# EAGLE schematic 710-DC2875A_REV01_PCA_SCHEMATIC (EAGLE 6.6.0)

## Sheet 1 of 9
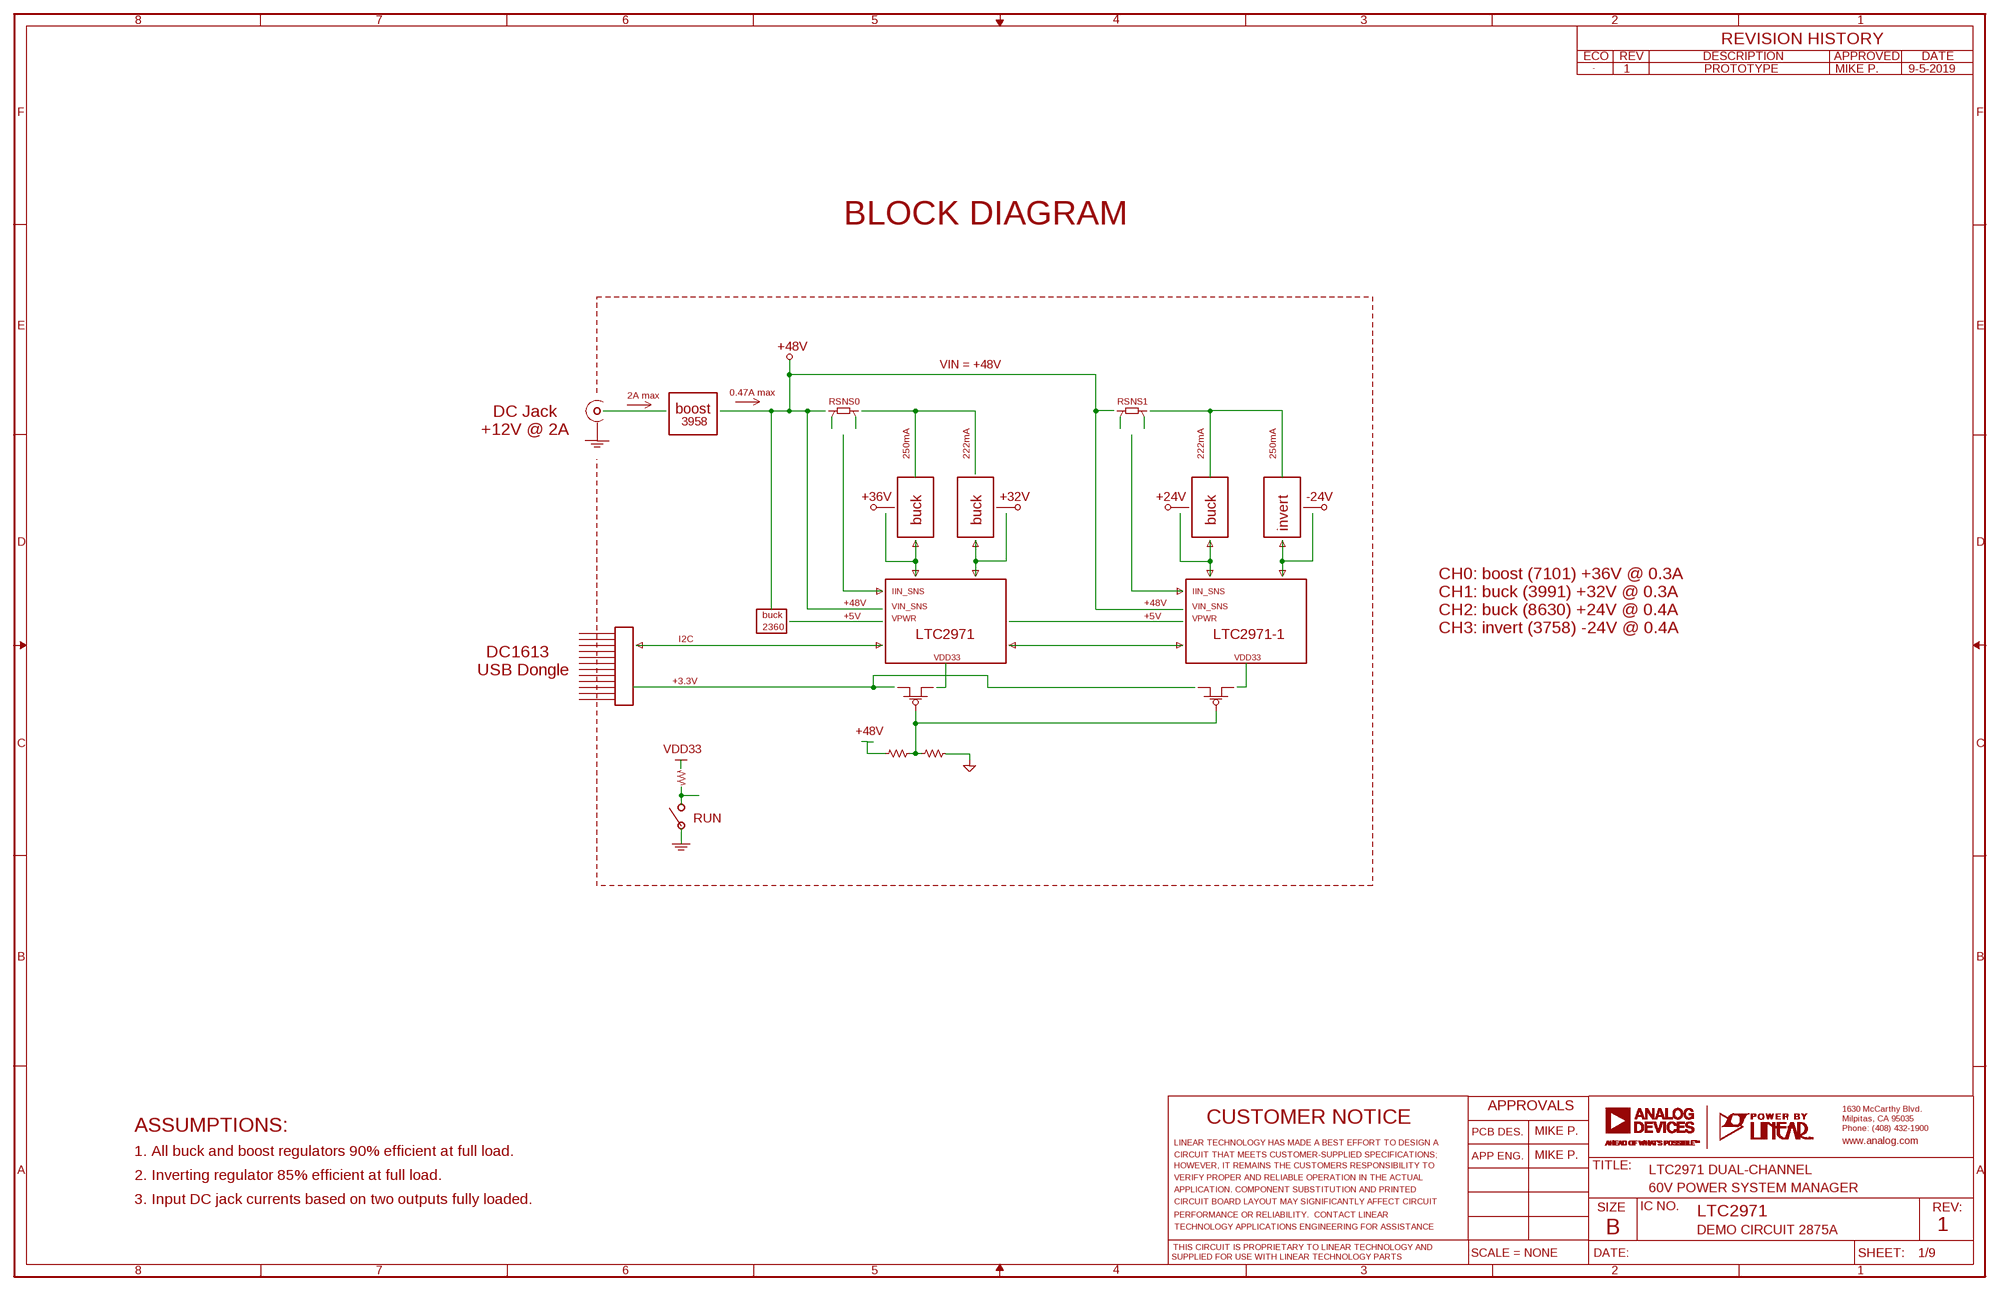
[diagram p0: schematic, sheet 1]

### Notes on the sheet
- 1 | PROTOTYPE | MIKE P. | 9-5-2019
- BLOCK DIAGRAM
- +48V
- VIN = +48V
- 0.47A max
- 2A max
- RSNS0 | RSNS1
- boost
- 3958
- DC Jack
  +12V @ 2A
- 250mA | 222mA | 222mA | 250mA
- +36V | +32V | +24V | -24V
- buck | buck | buck
- invert
- IIN_SNS | IIN_SNS
- +48V | +48V
- VIN_SNS | VIN_SNS
- buck | +5V | +5V
- VPWR | VPWR
- 2360
- CH0: boost (7101) +36V @ 0.3A
  CH1: buck (3991) +32V @ 0.3A
  CH2: buck (8630) +24V @ 0.4A
  CH3: invert (3758) -24V @ 0.4A
- LTC2971 | LTC2971-1
- I2C
- VDD33 | VDD33
- DC1613
  USB Dongle
- +3.3V
- +48V
- VDD33
- RUN
- ASSUMPTIONS: | MIKE P.
- 1. All buck and boost regulators 90% efficient at full load. | MIKE P.
- LTC2971 DUAL-CHANNEL
- 2. Inverting regulator 85% efficient at full load.
- 60V POWER SYSTEM MANAGER
- 3. Input DC jack currents based on two outputs fully loaded.
- LTC2971
- DEMO CIRCUIT 2875A | 1

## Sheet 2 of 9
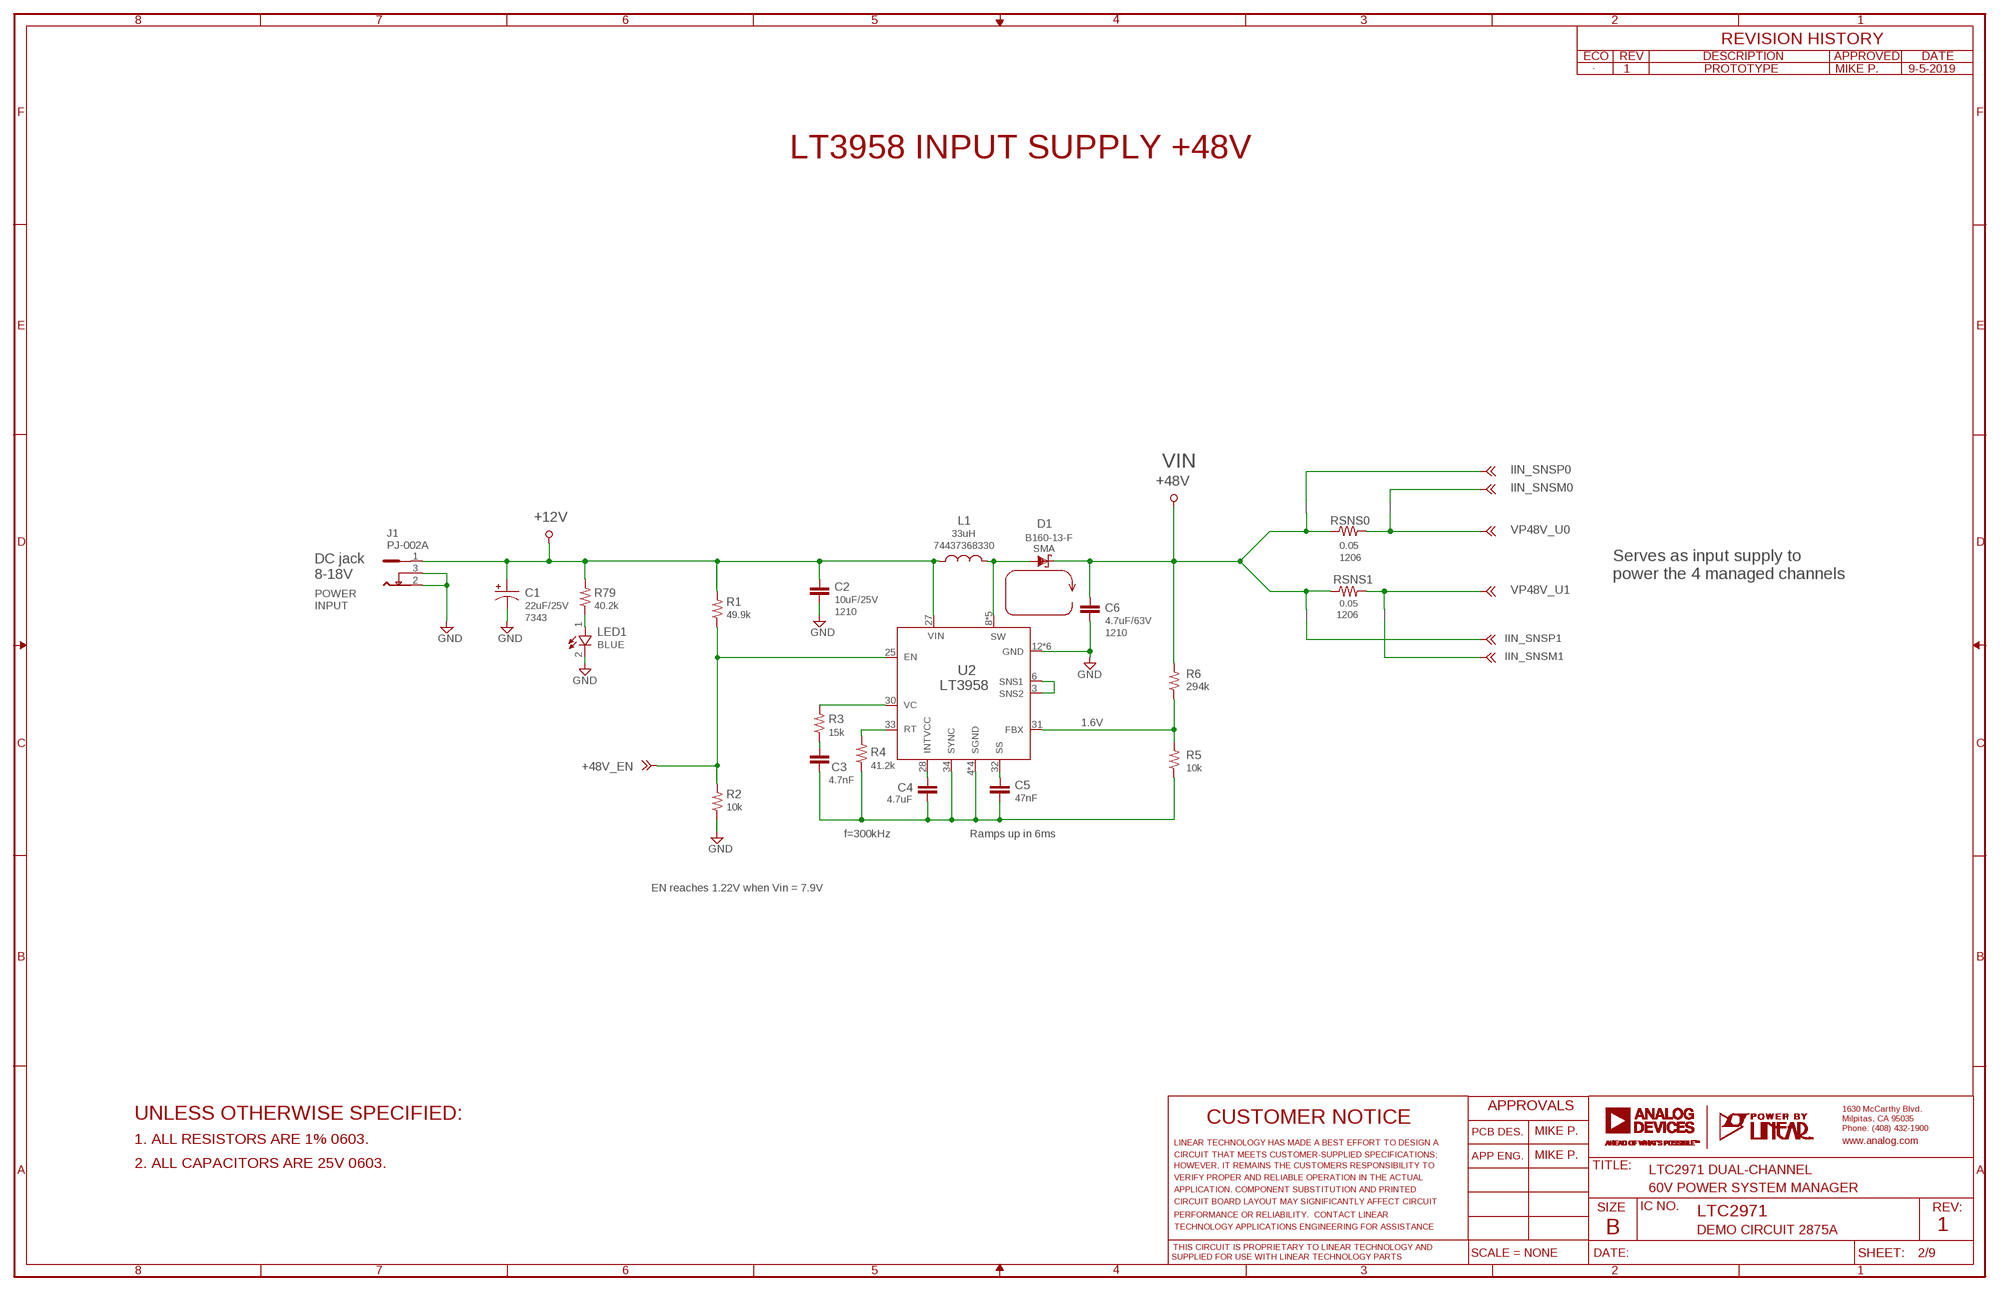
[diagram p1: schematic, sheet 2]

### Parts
C1  22uF/25V  CPOL-US7343  [C7343]
C2  10uF/25V  CC1210_BOX  [C1210_BOX]
C3  4.7nF  CC0603_BOX  [C0603_BOX]
C4  4.7uF  CC0603_BOX  [C0603_BOX]
C5  47nF  CC0603_BOX  [C0603_BOX]
C6  4.7uF/63V  CC1210_BOX  [C1210_BOX]
D1  B160-13-F  SCHOTTKY-DIODESMA  [SMA]
J1  PJ-002A  [PJ-002A/B]
L1  33uH  LWE-LHMI-10  [WE-LHMI-10]
LED1  BLUE  LED-0603  [CHIPLED_0603]
NB12  NODE_BREAKER_BOT  [NODE_BREAKER_BOT]
NB13  NODE_BREAKER_BOT  [NODE_BREAKER_BOT]
NB17  NODE_BREAKER_BOT  [NODE_BREAKER_BOT]
NB18  NODE_BREAKER_BOT  [NODE_BREAKER_BOT]
R1  49.9k  RR0603_BOX  [R0603_BOX]
R2  10k  RR0603_BOX  [R0603_BOX]
R3  15k  RR0603_BOX  [R0603_BOX]
R4  41.2k  RR0603_BOX  [R0603_BOX]
R5  10k  RR0603_BOX  [R0603_BOX]
R6  294k  RR0603_BOX  [R0603_BOX]
R79  40.2k  RR0603_BOX  [R0603_BOX]
RSNS0  0.05  RR1206_BOX  [R1206_BOX]
RSNS1  0.05  RR1206_BOX  [R1206_BOX]
TP14  +12V  TURRET_LARGE_2501  [TURRET_LARGE_2501]
TP15  +48V  TURRET_LARGE_2501  [TURRET_LARGE_2501]
TP36  TESPOINT_SMD  TESTPOINT_SMDVIA  [VIA]
U2  LT3958  [QFN36-5X6]

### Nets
+12V: C1.+ C2.1 J1.1 L1.1 R1.2 R79.2 TP14.TP U2.27(VIN) ; also sheet 9
+48V [HV]: C6.1 D1.C NB12.1 NB17.1 R6.2 RSNS0.1 RSNS1.1 TP15.TP ; also sheet 5
+48V_EN: R1.1 R2.2 TP36.1 U2.25(EN)
GND: C1.- C2.2 C6.2 J1.2 J1.3 LED1.C R2.1 U2.12(GND) U2.13(GND) U2.14(GND) U2.15(GND) U2.16(GND) U2.17(GND) ; also sheet 3,4,5,6,7,8,9
IIN_SNSM0 [HV]: NB13.2 ; also sheet 5
IIN_SNSM1 [HV]: NB18.2 ; also sheet 8
IIN_SNSP0 [HV]: NB12.2 ; also sheet 5
IIN_SNSP1 [HV]: NB17.2 ; also sheet 8
N$8: C4.1 U2.28(INTVCC)
N$12: LED1.A R79.1
N$13: U2.3(SNS2) U2.6(SNS1)
N$18: R3.2 U2.30(VC)
N$21: C5.1 U2.32(SS)
N$30 [HV]: D1.A L1.2 U2.8(SW) U2.9(SW) U2.20(SW) U2.21(SW) U2.38(SW)
N$32: R4.2 U2.33(RT)
N$51: R5.2 R6.1 U2.31(FBX)
N$61: C3.1 R3.1
SGND: C3.2 C4.2 C5.2 R4.1 R5.1 U2.4(SGND) U2.23(SGND) U2.24(SGND) U2.34(SYNC) U2.37(SGND)
VP48V_U0 [HV]: NB13.1 RSNS0.2 ; also sheet 3,4,5
VP48V_U1 [HV]: NB18.1 RSNS1.2 ; also sheet 6,7,8

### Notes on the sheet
- 1 | PROTOTYPE | MIKE P. | 9-5-2019
- LT3958 INPUT SUPPLY +48V
- VIN
- 74437368330
- SMA
- 1206
- DC jack
  8-18V
- Serves as input supply to 
  power the 4 managed channels
- POWER
  INPUT
- 1210
- 1206
- 7343
- 1210
- 1.6V
- f=300kHz | Ramps up in 6ms
- EN reaches 1.22V when Vin = 7.9V
- UNLESS OTHERWISE SPECIFIED:
- MIKE P.
- 1. ALL RESISTORS ARE 1% 0603.
- MIKE P.
- 2. ALL CAPACITORS ARE 25V 0603.
- LTC2971 DUAL-CHANNEL
- 60V POWER SYSTEM MANAGER
- LTC2971
- DEMO CIRCUIT 2875A | 1

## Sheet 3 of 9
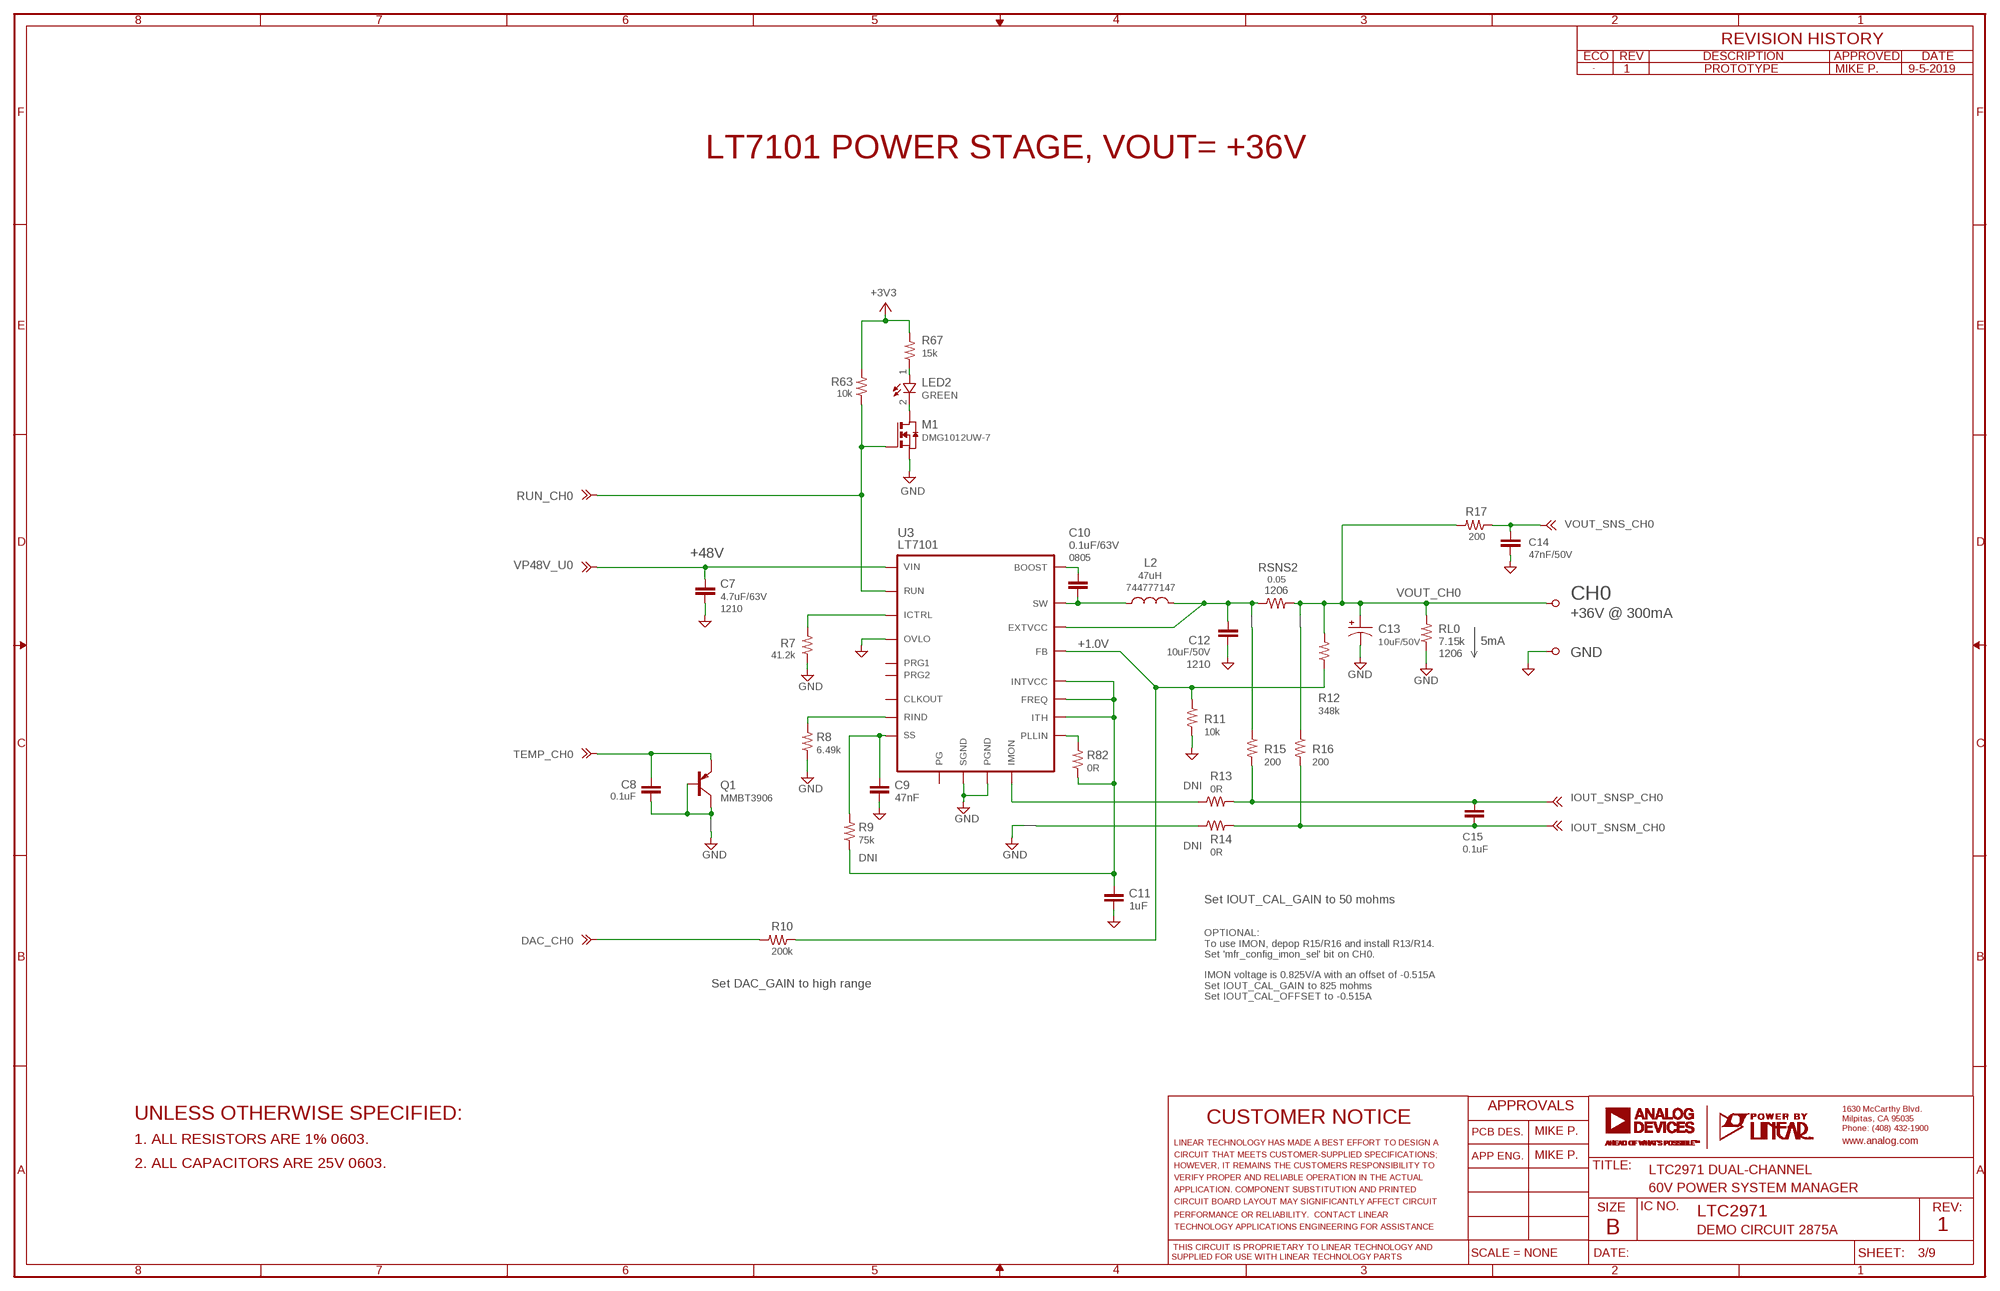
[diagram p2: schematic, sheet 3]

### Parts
C7  4.7uF/63V  CC1210_BOX  [C1210_BOX]
C8  0.1uF  CC0603_BOX  [C0603_BOX]
C9  47nF  CC0603_BOX  [C0603_BOX]
C10  0.1uF/63V  CC0805_BOX  [C0805_BOX]
C11  1uF  CC0603_BOX  [C0603_BOX]
C12  10uF/50V  CC1210_BOX  [C1210_BOX]
C13  10uF/50V  CPOL-USUD-6,3X5,8  [UD-6,3X5,8_NICHICON]
C14  47nF/50V  CC0603_BOX  [C0603_BOX]
C15  0.1uF  CC0603_BOX  [C0603_BOX]
L2  47uH  LWE-PD-7.3  [WE-PD-7.3]
LED2  GREEN  LED-0603  [CHIPLED_0603]
M1  DMG1012UW-7  NCH(SOT323)  [SOT323]
NB5  NODE_BREAKER  [NODE_BREAKER]
NB19  NODE_BREAKER  [NODE_BREAKER]
NB20  NODE_BREAKER  [NODE_BREAKER]
NB21  NODE_BREAKER  [NODE_BREAKER]
Q1  MMBT3906  PNP  [SC70]
R7  41.2k  RR0603_BOX  [R0603_BOX]
R8  6.49k  RR0603_BOX  [R0603_BOX]
R9  75k  RR0603_BOX  [R0603_BOX]
R10  200k  RR0603_BOX  [R0603_BOX]
R11  10k  RR0603_BOX  [R0603_BOX]
R12  348k  RR0603_BOX  [R0603_BOX]
R13  0R  RR0603_BOX  [R0603_BOX]
R14  0R  RR0603_BOX  [R0603_BOX]
R15  200  RR0603_BOX  [R0603_BOX]
R16  200  RR0603_BOX  [R0603_BOX]
R17  200  RR0603_BOX  [R0603_BOX]
R63  10k  RR0603_BOX  [R0603_BOX]
R67  15k  RR0603_BOX  [R0603_BOX]
R82  0R  RR0603_BOX  [R0603_BOX]
RL0  7.15k  RR1206_BOX  [R1206_BOX]
RSNS2  0.05  RR1206_BOX  [R1206_BOX]
TP0  CH0  TURRET_LARGE_2501  [TURRET_LARGE_2501]
TP20  TURRET_SMALL_2308  [TURRET_SMALL_2308]
TP24  TESPOINT_SMD  TESTPOINT_SMDVIA  [VIA]
TP25  TESPOINT_SMD  TESTPOINT_SMDVIA  [VIA]
TP26  TESPOINT_SMD  TESTPOINT_SMDVIA  [VIA]
U3  LT7101  [QFN36-5X6-UHE]

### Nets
DAC_CH0: R10.2 TP26.1 ; also sheet 5
GND: C7.2 C9.2 C11.2 C12.2 C13.- C14.2 M1.2(S) NB5.1 NB19.2 R7.1 R8.1 R11.2 RL0.1 TP20.TP1 U3.6(SGND) U3.7(OVLO) U3.35(PGND) U3.36(PGND) U3.37(PGND) ; also sheet 2,4,5,6,7,8,9
INTVCC: C11.1 R9.1 R82.1 U3.9(ITH) U3.11(FREQ) U3.21(INTVCC)
IOUT_SNSM_CH0 [HV]: C15.2 R14.2 R16.2 ; also sheet 5
IOUT_SNSP_CH0 [HV]: C15.1 R13.2 R15.2 ; also sheet 5
N$4: R7.2 U3.16(ICTRL)
N$6: LED2.C M1.3(D)
N$7: LED2.A R67.1
N$20: R8.2 U3.8(RIND)
N$64: C8.2 NB5.2 Q1.1(B) Q1.3(C)
N$73: C9.1 R9.2 U3.15(SS)
N$75 [HV]: R13.1 U3.17(IMON)
N$78 [HV]: C12.1 L2.2 NB20.2 RSNS2.1 U3.20(EXTVCC)
N$94: NB20.1 R15.1
N$98 [HV]: NB19.1 R14.1
N$99: NB21.1 R16.1
N$100: C10.2 L2.1 U3.24(SW) U3.25(SW) U3.26(SW)
N$114: C10.1 U3.27(BOOST)
N$116: R82.2 U3.12(PLLIN)
RUN_CH0: M1.1(G) R63.1 TP24.1 U3.3(RUN) ; also sheet 5
TEMP_CH0: C8.1 Q1.2(E) TP25.1 ; also sheet 5
VDD33_A: R63.2 R67.2 ; supply symbol labelled +3V3 ; also sheet 4,5,6,9
VFB0: R10.1 R11.1 R12.1 U3.10(FB)
VOUT_CH0 [HV]: C13.+ NB21.2 R12.2 R17.2 RL0.2 RSNS2.2 TP0.TP
VOUT_SNS_CH0 [HV]: C14.1 R17.1 ; also sheet 5
VP48V_U0 [HV]: C7.1 U3.30(VIN) U3.31(VIN) U3.32(VIN) ; also sheet 2,4,5
Unconnected: U3.13(CLKOUT) U3.14(PGOOD) U3.18(PRG1) U3.19(PRG2)

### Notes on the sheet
- 1 | PROTOTYPE | MIKE P. | 9-5-2019
- LT7101 POWER STAGE, VOUT= +36V
- +48V
- 0805
- 744777147
- 1206
- CH0
- 1210
- +36V @ 300mA
- +1.0V | 5mA
- 1210 | 1206
- DNI
- DNI
- DNI
- Set IOUT_CAL_GAIN to 50 mohms
- OPTIONAL:
  To use IMON, depop R15/R16 and install R13/R14.
  Set 'mfr_config_imon_sel' bit on CH0.
- Set DAC_GAIN to high range
- IMON voltage is 0.825V/A with an offset of -0.515A
  Set IOUT_CAL_GAIN to 825 mohms
  Set IOUT_CAL_OFFSET to -0.515A
- UNLESS OTHERWISE SPECIFIED:
- MIKE P.
- 1. ALL RESISTORS ARE 1% 0603.
- MIKE P.
- 2. ALL CAPACITORS ARE 25V 0603.
- LTC2971 DUAL-CHANNEL
- 60V POWER SYSTEM MANAGER
- LTC2971
- DEMO CIRCUIT 2875A | 1

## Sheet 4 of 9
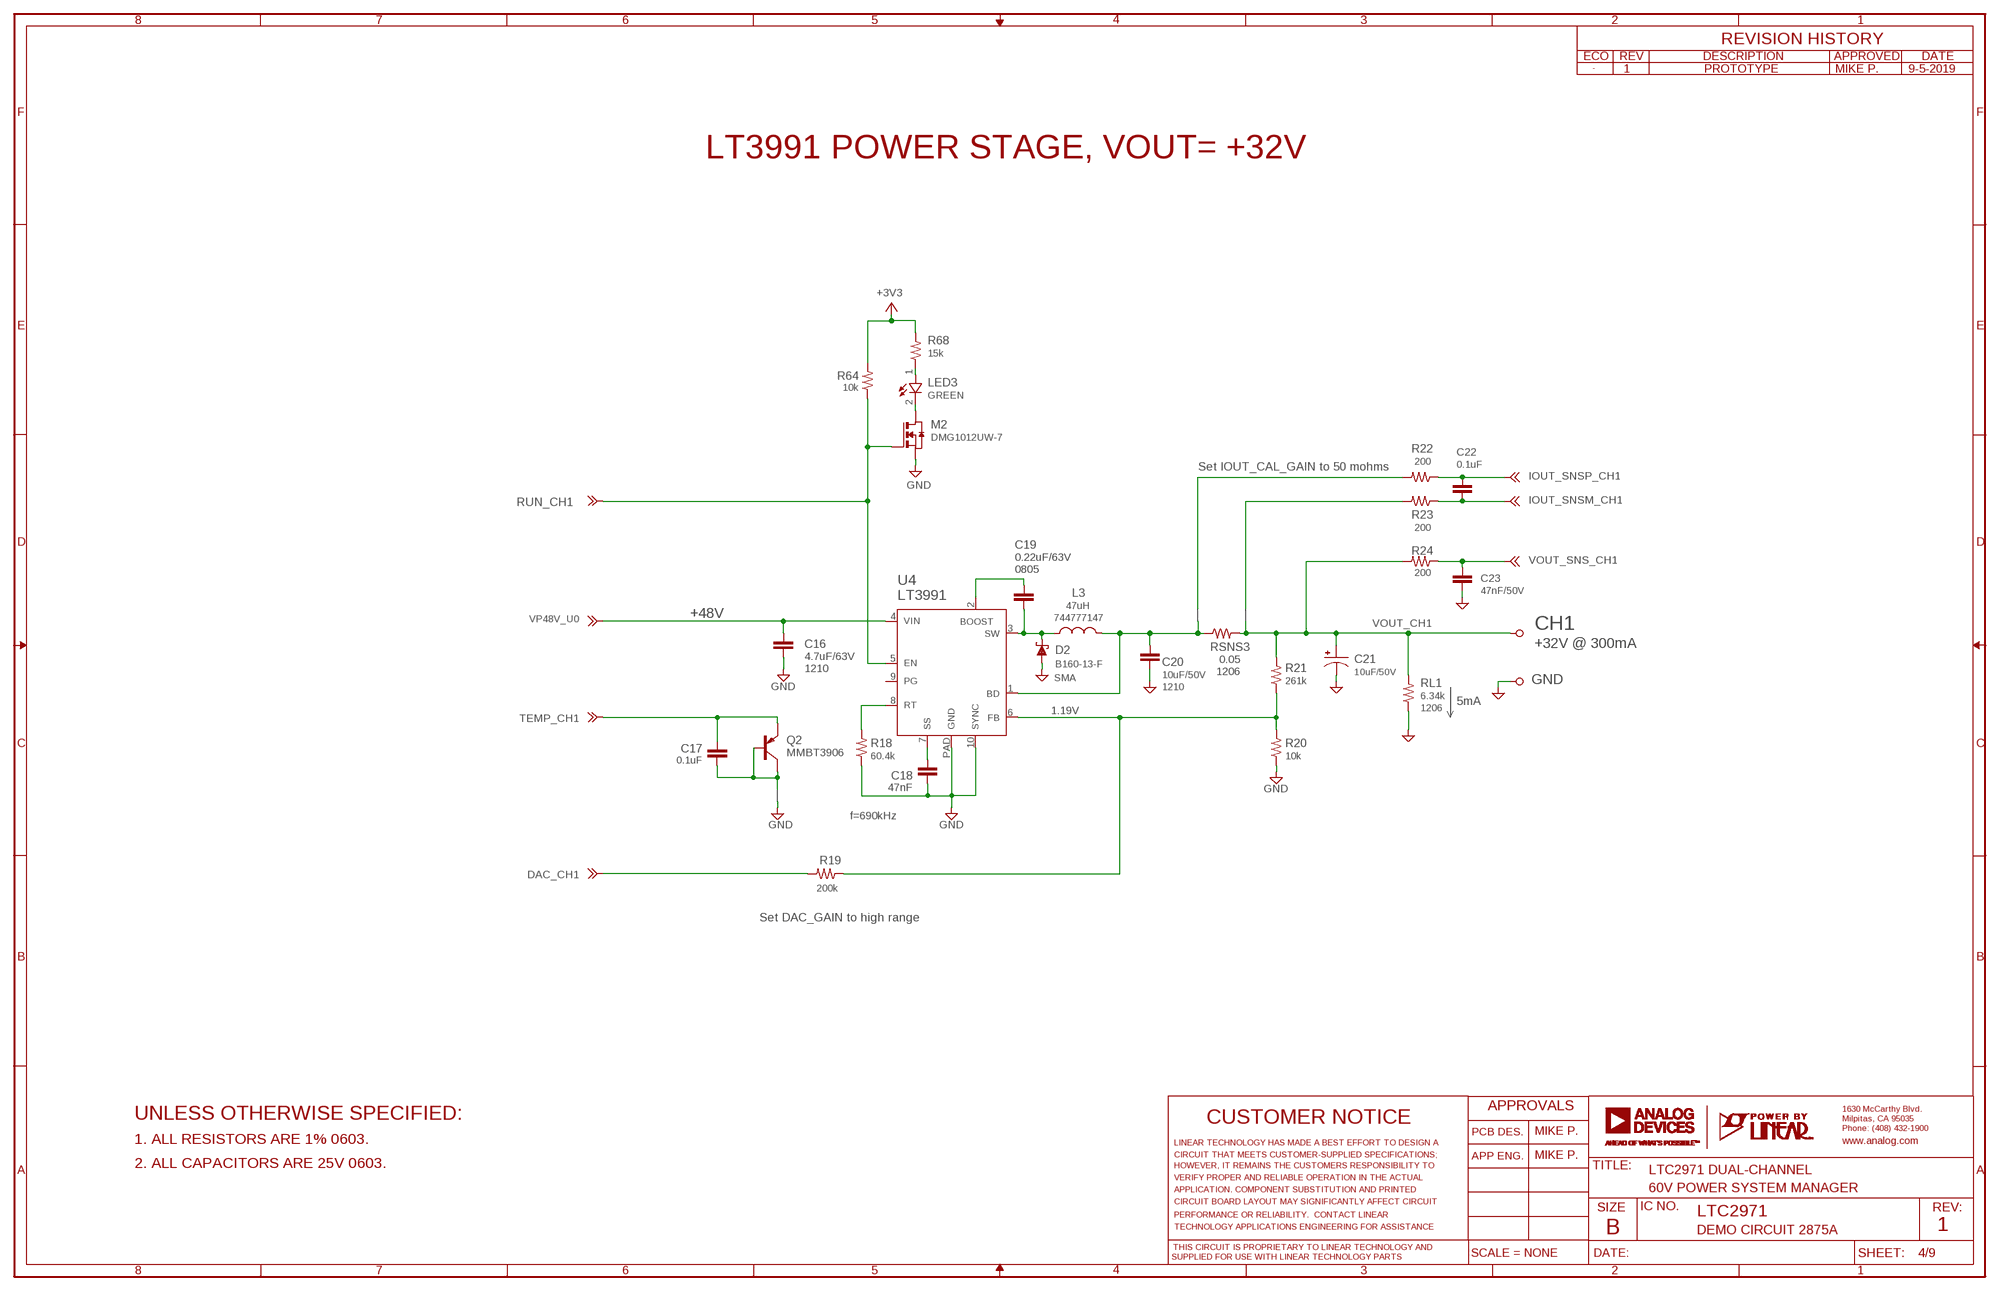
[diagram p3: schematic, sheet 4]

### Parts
C16  4.7uF/63V  CC1210_BOX  [C1210_BOX]
C17  0.1uF  CC0603_BOX  [C0603_BOX]
C18  47nF  CC0603_BOX  [C0603_BOX]
C19  0.22uF/63V  CC0805_BOX  [C0805_BOX]
C20  10uF/50V  CC1210_BOX  [C1210_BOX]
C21  10uF/50V  CPOL-USUD-6,3X5,8  [UD-6,3X5,8_NICHICON]
C22  0.1uF  CC0603_BOX  [C0603_BOX]
C23  47nF/50V  CC0603_BOX  [C0603_BOX]
D2  B160-13-F  SCHOTTKY-DIODESMA  [SMA]
L3  47uH  LWE-PD-7.3  [WE-PD-7.3]
LED3  GREEN  LED-0603  [CHIPLED_0603]
M2  DMG1012UW-7  NCH(SOT323)  [SOT323]
NB3  NODE_BREAKER  [NODE_BREAKER]
NB4  NODE_BREAKER  [NODE_BREAKER]
NB14  NODE_BREAKER  [NODE_BREAKER]
Q2  MMBT3906  PNP  [SC70]
R18  60.4k  RR0603_BOX  [R0603_BOX]
R19  200k  RR0603_BOX  [R0603_BOX]
R20  10k  RR0603_BOX  [R0603_BOX]
R21  261k  RR0603_BOX  [R0603_BOX]
R22  200  RR0603_BOX  [R0603_BOX]
R23  200  RR0603_BOX  [R0603_BOX]
R24  200  RR0603_BOX  [R0603_BOX]
R64  10k  RR0603_BOX  [R0603_BOX]
R68  15k  RR0603_BOX  [R0603_BOX]
RL1  6.34k  RR1206_BOX  [R1206_BOX]
RSNS3  0.05  RR1206_BOX  [R1206_BOX]
TP1  CH1  TURRET_LARGE_2501  [TURRET_LARGE_2501]
TP21  TURRET_SMALL_2308  [TURRET_SMALL_2308]
TP27  TESPOINT_SMD  TESTPOINT_SMDVIA  [VIA]
TP28  TESPOINT_SMD  TESTPOINT_SMDVIA  [VIA]
TP29  TESPOINT_SMD  TESTPOINT_SMDVIA  [VIA]
U4  LT3991  [MSOP10_EXP]

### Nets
DAC_CH1: R19.2 TP29.1 ; also sheet 5
GND: C16.2 C18.2 C20.2 C21.- C23.2 D2.A M2.2(S) NB14.1 R18.1 R20.1 RL1.1 TP21.TP1 U4.10(SYNC) U4.PAD(GND) ; also sheet 2,3,5,6,7,8,9
IOUT_SNSM_CH1 [HV]: C22.2 R23.1 ; also sheet 5
IOUT_SNSP_CH1 [HV]: C22.1 R22.1 ; also sheet 5
N$10: LED3.C M2.3(D)
N$11: LED3.A R68.1
N$33: R18.2 U4.8(RT)
N$36 [HV]: C20.1 L3.2 NB3.1 RSNS3.1 U4.1(BD)
N$59: C18.1 U4.7(SS)
N$67: C17.2 NB14.2 Q2.1(B) Q2.3(C)
N$70: C19.2 D2.C L3.1 U4.3(SW)
N$71: C19.1 U4.2(BOOST)
N$300 [HV]: NB3.2 R22.2
N$301 [HV]: NB4.2 R23.2
RUN_CH1: M2.1(G) R64.1 TP27.1 U4.5(EN) ; also sheet 5
TEMP_CH1: C17.1 Q2.2(E) TP28.1 ; also sheet 5
VDD33_A: R64.2 R68.2 ; supply symbol labelled +3V3 ; also sheet 3,5,6,9
VFB1: R19.1 R20.2 R21.1 U4.6(FB)
VOUT_CH1 [HV]: C21.+ NB4.1 R21.2 R24.2 RL1.2 RSNS3.2 TP1.TP
VOUT_SNS_CH1 [HV]: C23.1 R24.1 ; also sheet 5
VP48V_U0 [HV]: C16.1 U4.4(VIN) ; also sheet 2,3,5
Unconnected: U4.9(PG)

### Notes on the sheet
- 1 | PROTOTYPE | MIKE P. | 9-5-2019
- LT3991 POWER STAGE, VOUT= +32V
- Set IOUT_CAL_GAIN to 50 mohms
- 0805
- +48V
- 744777147
- CH1
- +32V @ 300mA
- 1210 | 1206
- SMA
- 1210
- 5mA
- 1206
- 1.19V
- f=690kHz
- Set DAC_GAIN to high range
- UNLESS OTHERWISE SPECIFIED:
- MIKE P.
- 1. ALL RESISTORS ARE 1% 0603.
- MIKE P.
- 2. ALL CAPACITORS ARE 25V 0603.
- LTC2971 DUAL-CHANNEL
- 60V POWER SYSTEM MANAGER
- LTC2971
- DEMO CIRCUIT 2875A | 1

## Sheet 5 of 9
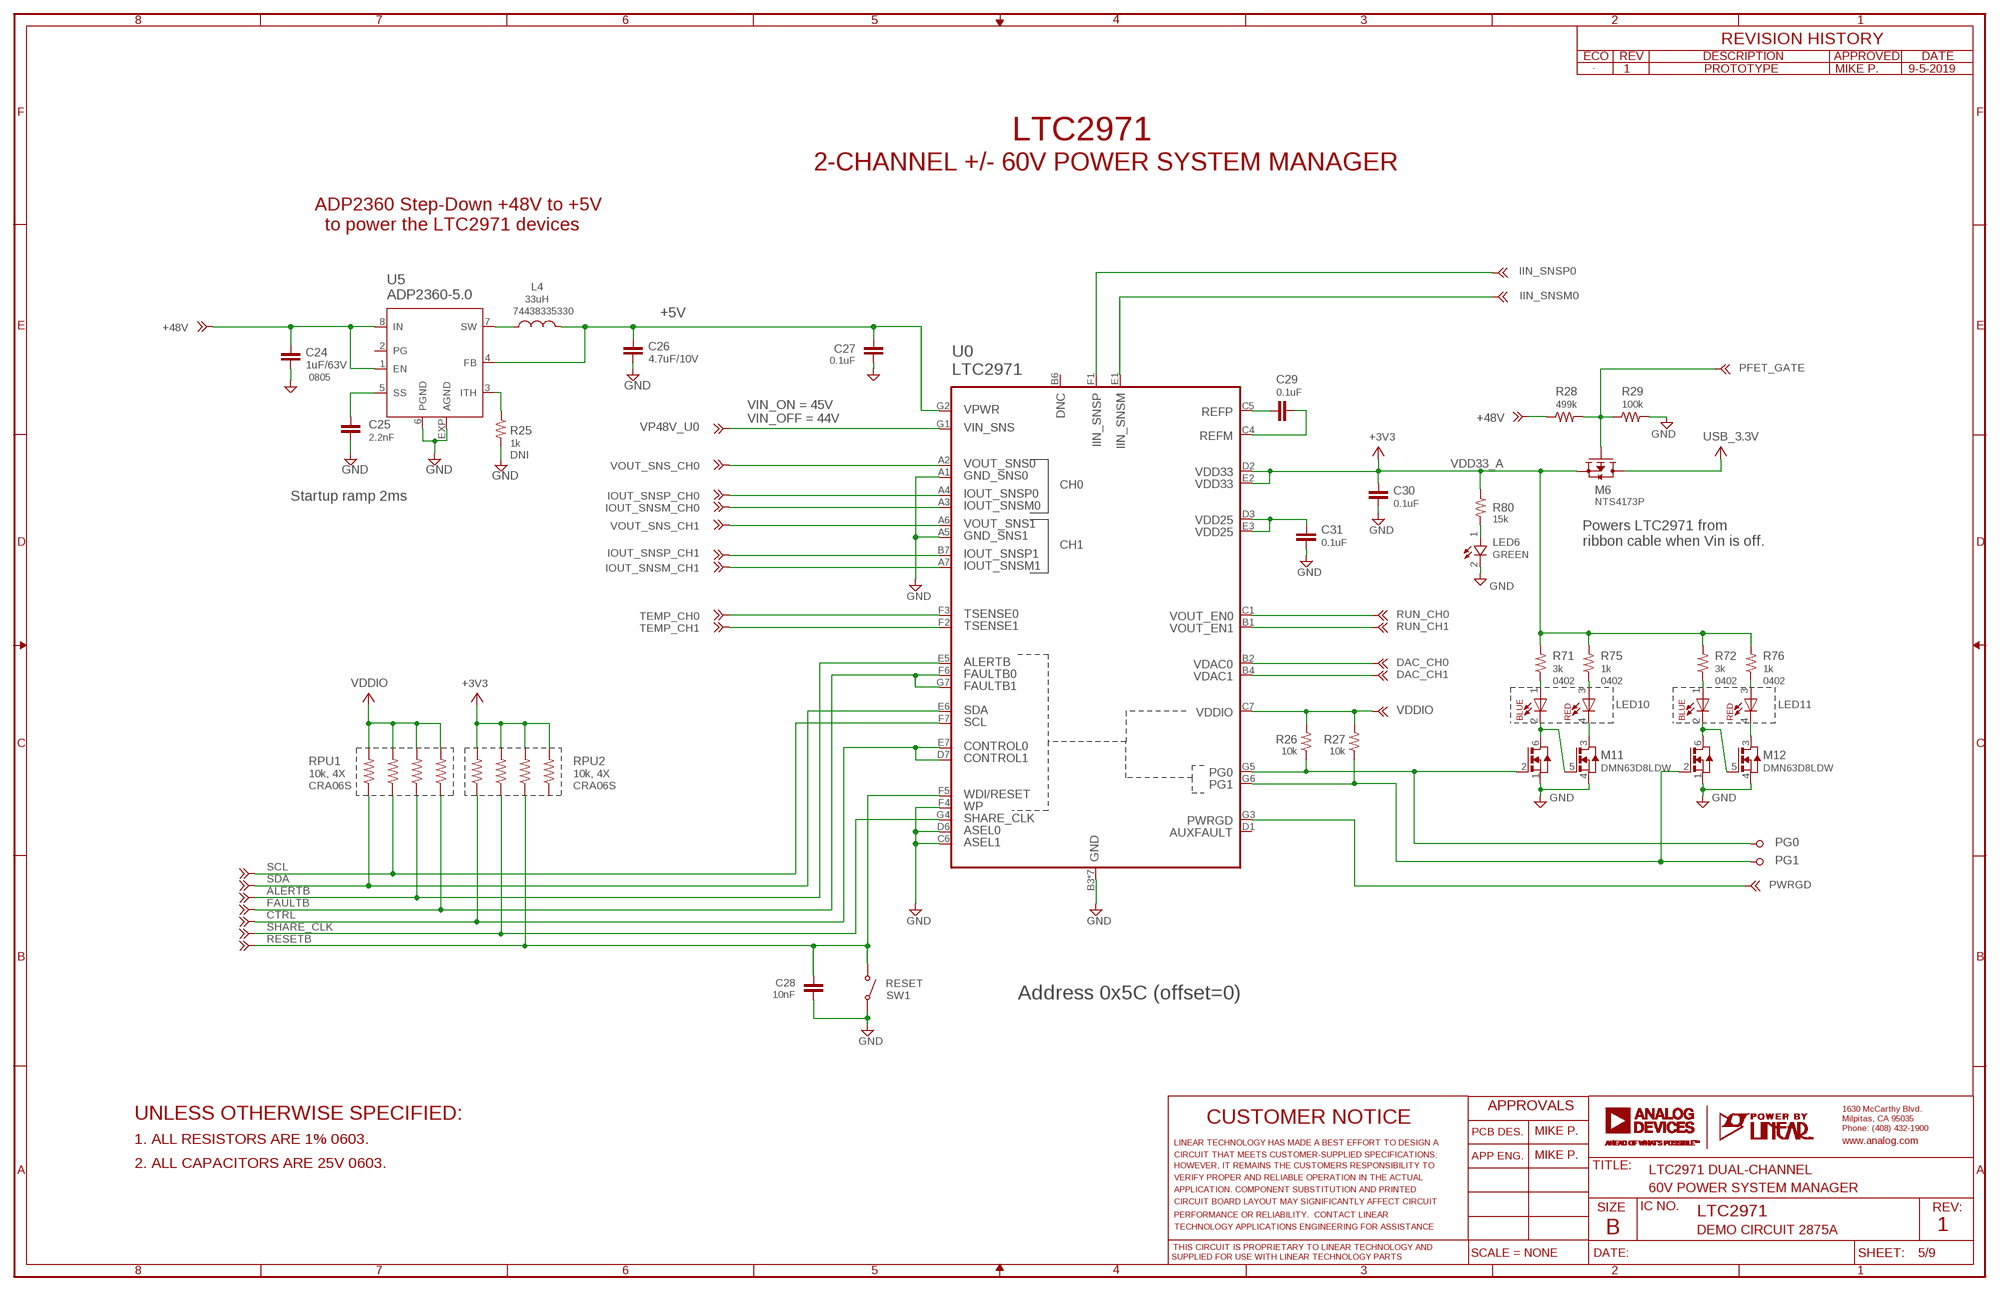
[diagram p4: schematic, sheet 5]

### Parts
C24  1uF/63V  CC0805_BOX  [C0805_BOX]
C25  2.2nF  CC0603_BOX  [C0603_BOX]
C26  4.7uF/10V  CC0603_BOX  [C0603_BOX]
C27  0.1uF  CC0603_BOX  [C0603_BOX]
C28  10nF  CC0603_BOX  [C0603_BOX]
C29  0.1uF  CC0603_BOX  [C0603_BOX]
C30  0.1uF  CC0603_BOX  [C0603_BOX]
C31  0.1uF  CC0603_BOX  [C0603_BOX]
L4  33uH  LWE-MAPI-3.0  [WE-MAPI-3015]
LED6  GREEN  LED-0603  [CHIPLED_0603]
LED10  LED-DUAL-COLOR-BL-RD  [LED-DUAL_1.6X0.8MM]
LED11  LED-DUAL-COLOR-BL-RD  [LED-DUAL_1.6X0.8MM]
M6  NTS4173P  PCH(SOT323)  [SOT323]
M11  DMN63D8LDW  NCH_DUAL_REVERSIBLE  [SOT-363]
M12  DMN63D8LDW  NCH_DUAL_REVERSIBLE  [SOT-363]
R25  1k  RR0603_BOX  [R0603_BOX]
R26  10k  RR0603_BOX  [R0603_BOX]
R27  10k  RR0603_BOX  [R0603_BOX]
R28  499k  RR0603_BOX  [R0603_BOX]
R29  100k  RR0603_BOX  [R0603_BOX]
R71  3k  RR0402_BOX  [R0402_BOX]
R72  3k  RR0402_BOX  [R0402_BOX]
R75  1k  RR0402_BOX  [R0402_BOX]
R76  1k  RR0402_BOX  [R0402_BOX]
R80  15k  RR0603_BOX  [R0603_BOX]
RPU1  10k, 4X  R_ARRAY_4X_CRA06S  [R_VISHAY_CRA06S]
RPU2  10k, 4X  R_ARRAY_4X_CRA06S  [R_VISHAY_CRA06S]
SW1  RS-282G05A3-SM RT  SWITCH_PTS635  [SWITCH_PTS635]
TP16  PG1  TURRET_SMALL_2308  [TURRET_SMALL_2308]
TP17  PG0  TURRET_SMALL_2308  [TURRET_SMALL_2308]
U0  LTC2971  [BGA49]
U5  ADP2360-5.0  ADP2360  [LFCSP8]

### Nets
+48V [HV]: C24.1 R28.1 U5.1(EN) U5.8(VIN) ; also sheet 2
ALERTB: RPU1.R3_1 U0.E5(ALERTB) ; also sheet 8,9
CTRL: RPU2.R1_1 U0.D7(CTRL1) U0.E7(CTRL0) ; also sheet 8,9
DAC_CH0: U0.B2(VDAC0) ; also sheet 3
DAC_CH1: U0.B4(VDAC1) ; also sheet 4
FAULTB: RPU1.R4_1 U0.F6(FAULTB0) U0.G7(FAULTB1) ; also sheet 8,9
GND: C24.2 C25.2 C26.2 C27.1 C28.1 C30.2 C31.1 LED6.C M11.1(S1) M11.4(S2) M12.1(S1) M12.4(S2) R25.2 R29.2 SW1.SW2 U0.A1(GND_SNS0) U0.A5(GND_SNS1) U0.B3(GND) U0.B5(GND) U0.C2(GND) U0.C3(GND) U0.C6(ASEL1) U0.D4(GND) U0.D5(GND) U0.D6(ASEL0) U0.E4(GND) U0.F4(WP) U5.6(PGND) U5.EXP(AGND) ; also sheet 2,3,4,6,7,8,9
IIN_SNSM0 [HV]: U0.E1(IIN_SNSM) ; also sheet 2
IIN_SNSP0 [HV]: U0.F1(IIN_SNSP) ; also sheet 2
IOUT_SNSM_CH0 [HV]: U0.A3(IOUT_SNSM0) ; also sheet 3
IOUT_SNSM_CH1 [HV]: U0.A7(IOUT_SNSM1) ; also sheet 4
IOUT_SNSP_CH0 [HV]: U0.A4(IOUT_SNSP0) ; also sheet 3
IOUT_SNSP_CH1 [HV]: U0.B7(IOUT_SNSP1) ; also sheet 4
N$23: C25.1 U5.5(SS)
N$28: LED11.2(C2) M12.5(G2) M12.6(D1)
N$46: L4.1 U5.7(SW)
N$48: R25.1 U5.3(ITH)
N$49: C29.2 U0.C4(REFM)
N$52: C31.2 U0.D3(VDD25_IO) U0.E3(VDD25_IN)
N$53: C29.1 U0.C5(REFP)
N$56: LED11.1(A1) R72.1
N$57: LED11.4(C4) M12.3(D2)
N$58: LED10.1(A1) R71.1
N$60: LED10.3(A3) R75.1
N$63: LED6.A R80.2
N$82: LED10.2(C2) M11.5(G2) M11.6(D1)
N$83: LED11.3(A3) R76.1
N$96: LED10.4(C4) M11.3(D2)
PFET_GATE: M6.1(G) R28.2 R29.1 ; also sheet 8
PG0: M11.2(G1) R26.1 TP16.TP1 U0.G5(PG0)
PG1: M12.2(G1) R27.1 TP17.TP1 U0.G6(PG1)
PWRGD: U0.G3(PWRGD) ; also sheet 8,9
RESETB: C28.2 RPU2.R3_1 SW1.SW1 U0.F5(WDI-RESET) ; also sheet 8,9
RUN_CH0: U0.C1(VOUT_EN0) ; also sheet 3
RUN_CH1: U0.B1(VOUT_EN1) ; also sheet 4
SCL: RPU1.R2_1 U0.F7(SCL) ; also sheet 8,9
SDA: RPU1.R1_1 U0.E6(SDA) ; also sheet 8,9
SHARE_CLK: RPU2.R2_1 U0.G4(SHARE_CLK) ; also sheet 8,9
TEMP_CH0: U0.F3(TSENSE0) ; also sheet 3
TEMP_CH1: U0.F2(TSENSE1) ; also sheet 4
USB_3.3V: M6.3(D) ; supply symbol labelled +3V3 ; also sheet 8,9
VDD33_A: C30.1 M6.2(S) R71.2 R72.2 R75.2 R76.2 R80.1 RPU2.R1_2 RPU2.R2_2 RPU2.R3_2 RPU2.R4_2 U0.D2(VDD33_IO) U0.E2(VDD33_IN) ; supply symbol labelled +3V3 ; also sheet 3,4,6,9
VDDIO: R26.2 R27.2 RPU1.R1_2 RPU1.R2_2 RPU1.R3_2 RPU1.R4_2 U0.C7(VDDIO) ; supply symbol labelled +3V3 ; also sheet 8,9
VOUT_SNS_CH0 [HV]: U0.A2(VOUT_SNS0) ; also sheet 3
VOUT_SNS_CH1 [HV]: U0.A6(VOUT_SNS1) ; also sheet 4
VP5P0: C26.1 C27.2 L4.2 U0.G2(VPWR) U5.4(FB) ; also sheet 8
VP48V_U0 [HV]: U0.G1(VIN_SNS) ; also sheet 2,3,4
Unconnected: RPU2.R4_1 U0.B6(DNC) U0.D1(AUXFAULT) U5.2(PG)

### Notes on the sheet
- 1 | PROTOTYPE | MIKE P. | 9-5-2019
- LTC2971
- 2-CHANNEL +/- 60V POWER SYSTEM MANAGER
- ADP2360 Step-Down +48V to +5V
    to power the LTC2971 devices
- 74438335330
- +5V
- 0805
- VIN_ON = 45V
  VIN_OFF = 44V
- DNI
- Startup ramp 2ms
- Powers LTC2971 from 
  ribbon cable when Vin is off.
- 0402 | 0402 | 0402 | 0402
- CRA06S | CRA06S
- RESET
- Address 0x5C (offset=0)
- UNLESS OTHERWISE SPECIFIED:
- MIKE P.
- 1. ALL RESISTORS ARE 1% 0603.
- MIKE P.
- 2. ALL CAPACITORS ARE 25V 0603.
- LTC2971 DUAL-CHANNEL
- 60V POWER SYSTEM MANAGER
- LTC2971
- DEMO CIRCUIT 2875A | 1

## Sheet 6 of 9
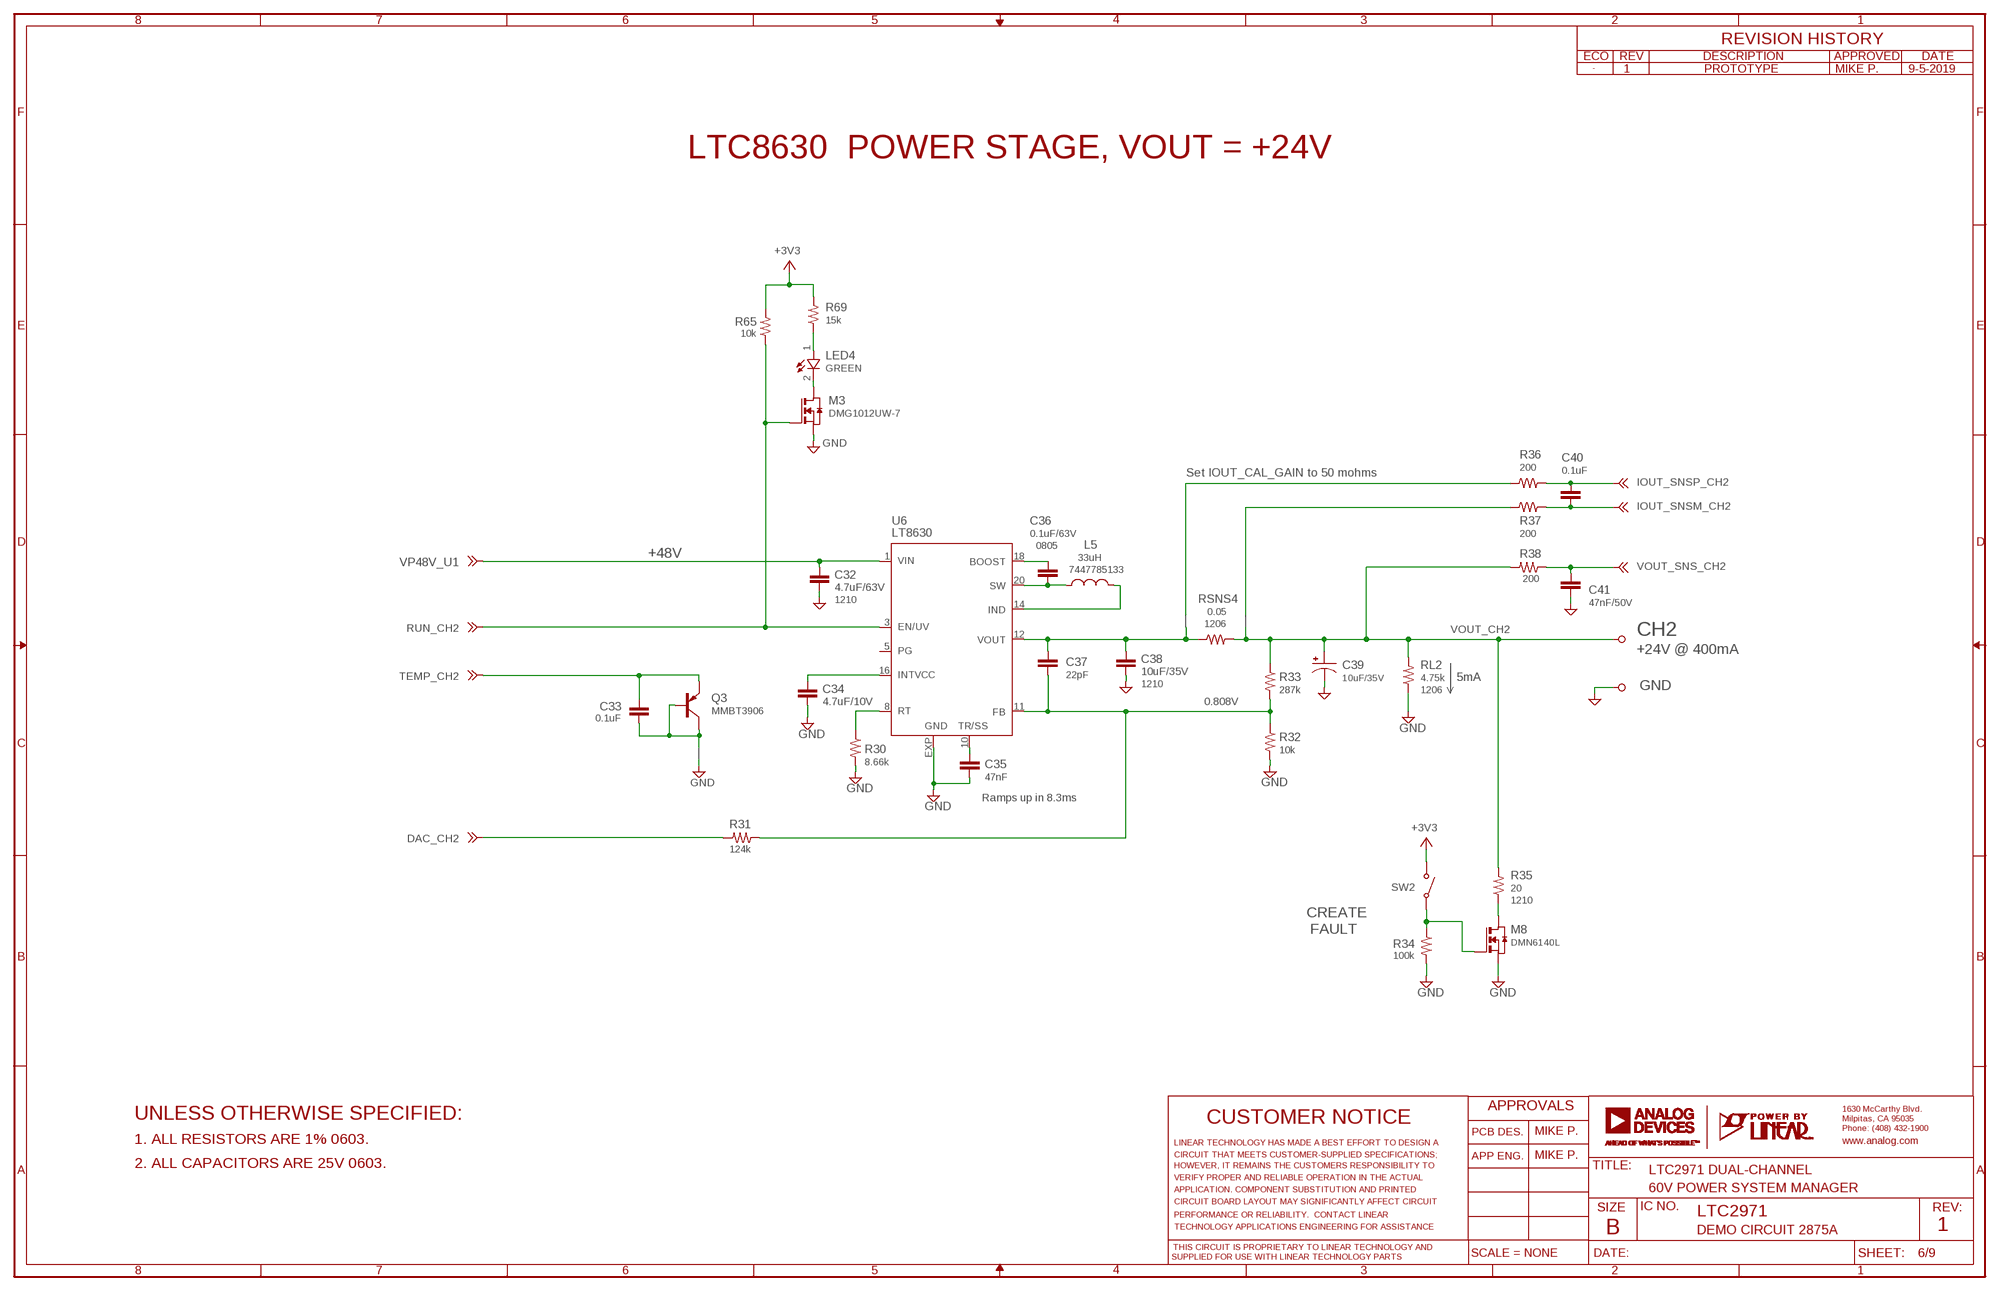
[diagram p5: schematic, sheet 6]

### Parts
C32  4.7uF/63V  CC1210_BOX  [C1210_BOX]
C33  0.1uF  CC0603_BOX  [C0603_BOX]
C34  4.7uF/10V  CC0603_BOX  [C0603_BOX]
C35  47nF  CC0603_BOX  [C0603_BOX]
C36  0.1uF/63V  CC0805_BOX  [C0805_BOX]
C37  22pF  CC0603_BOX  [C0603_BOX]
C38  10uF/35V  CC1210_BOX  [C1210_BOX]
C39  10uF/35V  CPOL-USUD-6,3X5,8  [UD-6,3X5,8_NICHICON]
C40  0.1uF  CC0603_BOX  [C0603_BOX]
C41  47nF/50V  CC0603_BOX  [C0603_BOX]
L5  33uH  LWE-PD-6.0  [WE-PD-6.0]
LED4  GREEN  LED-0603  [CHIPLED_0603]
M3  DMG1012UW-7  NCH(SOT323)  [SOT323]
M8  DMN6140L  NCH(SOT23)  [SOT23]
NB1  NODE_BREAKER  [NODE_BREAKER]
NB2  NODE_BREAKER  [NODE_BREAKER]
NB15  NODE_BREAKER  [NODE_BREAKER]
Q3  MMBT3906  PNP  [SC70]
R30  8.66k  RR0603_BOX  [R0603_BOX]
R31  124k  RR0603_BOX  [R0603_BOX]
R32  10k  RR0603_BOX  [R0603_BOX]
R33  287k  RR0603_BOX  [R0603_BOX]
R34  100k  RR0603_BOX  [R0603_BOX]
R35  20  RR1210_BOX  [R1210_BOX]
R36  200  RR0603_BOX  [R0603_BOX]
R37  200  RR0603_BOX  [R0603_BOX]
R38  200  RR0603_BOX  [R0603_BOX]
R65  10k  RR0603_BOX  [R0603_BOX]
R69  15k  RR0603_BOX  [R0603_BOX]
RL2  4.75k  RR1206_BOX  [R1206_BOX]
RSNS4  0.05  RR1206_BOX  [R1206_BOX]
SW2  RS-282G05A3-SM RT  SWITCH_PTS635  [SWITCH_PTS635]
TP2  CH2  TURRET_LARGE_2501  [TURRET_LARGE_2501]
TP22  TURRET_SMALL_2308  [TURRET_SMALL_2308]
TP30  TESTPOINT_SMD  TESTPOINT_SMDVIA  [VIA]
TP31  TESPOINT_SMD  TESTPOINT_SMDVIA  [VIA]
TP32  TESPOINT_SMD  TESTPOINT_SMDVIA  [VIA]
U6  LT8630  [TSSOP20EXP_HV]

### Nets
DAC_CH2: R31.2 TP32.1 ; also sheet 8
GND: C32.2 C34.2 C35.2 C38.2 C39.- C41.2 M3.2(S) M8.2(S) NB15.1 R30.2 R32.2 R34.2 RL2.1 TP22.TP1 U6.EXP(GND) ; also sheet 2,3,4,5,7,8,9
IOUT_SNSM_CH2: C40.2 R37.2 ; also sheet 8
IOUT_SNSP_CH2: C40.1 R36.2 ; also sheet 8
N$2: M8.1(G) R34.1 SW2.SW2
N$5: LED4.C M3.3(D)
N$9: LED4.A R69.1
N$27: C37.1 C38.1 NB1.1 RSNS4.1 U6.12(VOUT)
N$35 [HV]: C36.1 U6.18(BOOST)
N$37: C34.1 U6.16(INTVCC)
N$38: R30.1 U6.8(RT)
N$39 [HV]: C36.2 L5.1 U6.20(SW)
N$40: L5.2 U6.14(IND)
N$41: C35.1 U6.10(TR/SS)
N$55: M8.3(D) R35.1
N$68: C33.2 NB15.2 Q3.1(B) Q3.3(C)
N$109: NB1.2 R36.1
N$500: NB2.2 R37.1
RUN_CH2: M3.1(G) R65.1 TP30.1 U6.3(EN/UV) ; also sheet 8
TEMP_CH2: C33.1 Q3.2(E) TP31.1 ; also sheet 8
VDD33_A: SW2.SW1 ; supply symbol labelled +3V3 ; also sheet 3,4,5,9
VDD33_B: R65.2 R69.2 ; supply symbol labelled +3V3 ; also sheet 7,8
VFB2: C37.2 R31.1 R32.1 R33.2 U6.11(FB)
VOUT_CH2: C39.+ NB2.1 R33.1 R35.2 R38.2 RL2.2 RSNS4.2 TP2.TP
VOUT_SNS_CH2: C41.1 R38.1 ; also sheet 8
VP48V_U1 [HV]: C32.1 U6.1(VIN) ; also sheet 2,7,8
Unconnected: U6.5(PG)

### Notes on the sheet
- 1 | PROTOTYPE | MIKE P. | 9-5-2019
- LTC8630  POWER STAGE, VOUT = +24V
- Set IOUT_CAL_GAIN to 50 mohms
- 0805
- +48V
- 7447785133
- 1210
- 1206
- CH2
- +24V @ 400mA
- 5mA
- 1210
- 1206
- 0.808V
- Ramps up in 8.3ms
- 1210
- CREATE
   FAULT
- UNLESS OTHERWISE SPECIFIED:
- MIKE P.
- 1. ALL RESISTORS ARE 1% 0603.
- MIKE P.
- 2. ALL CAPACITORS ARE 25V 0603.
- LTC2971 DUAL-CHANNEL
- 60V POWER SYSTEM MANAGER
- LTC2971
- DEMO CIRCUIT 2875A | 1

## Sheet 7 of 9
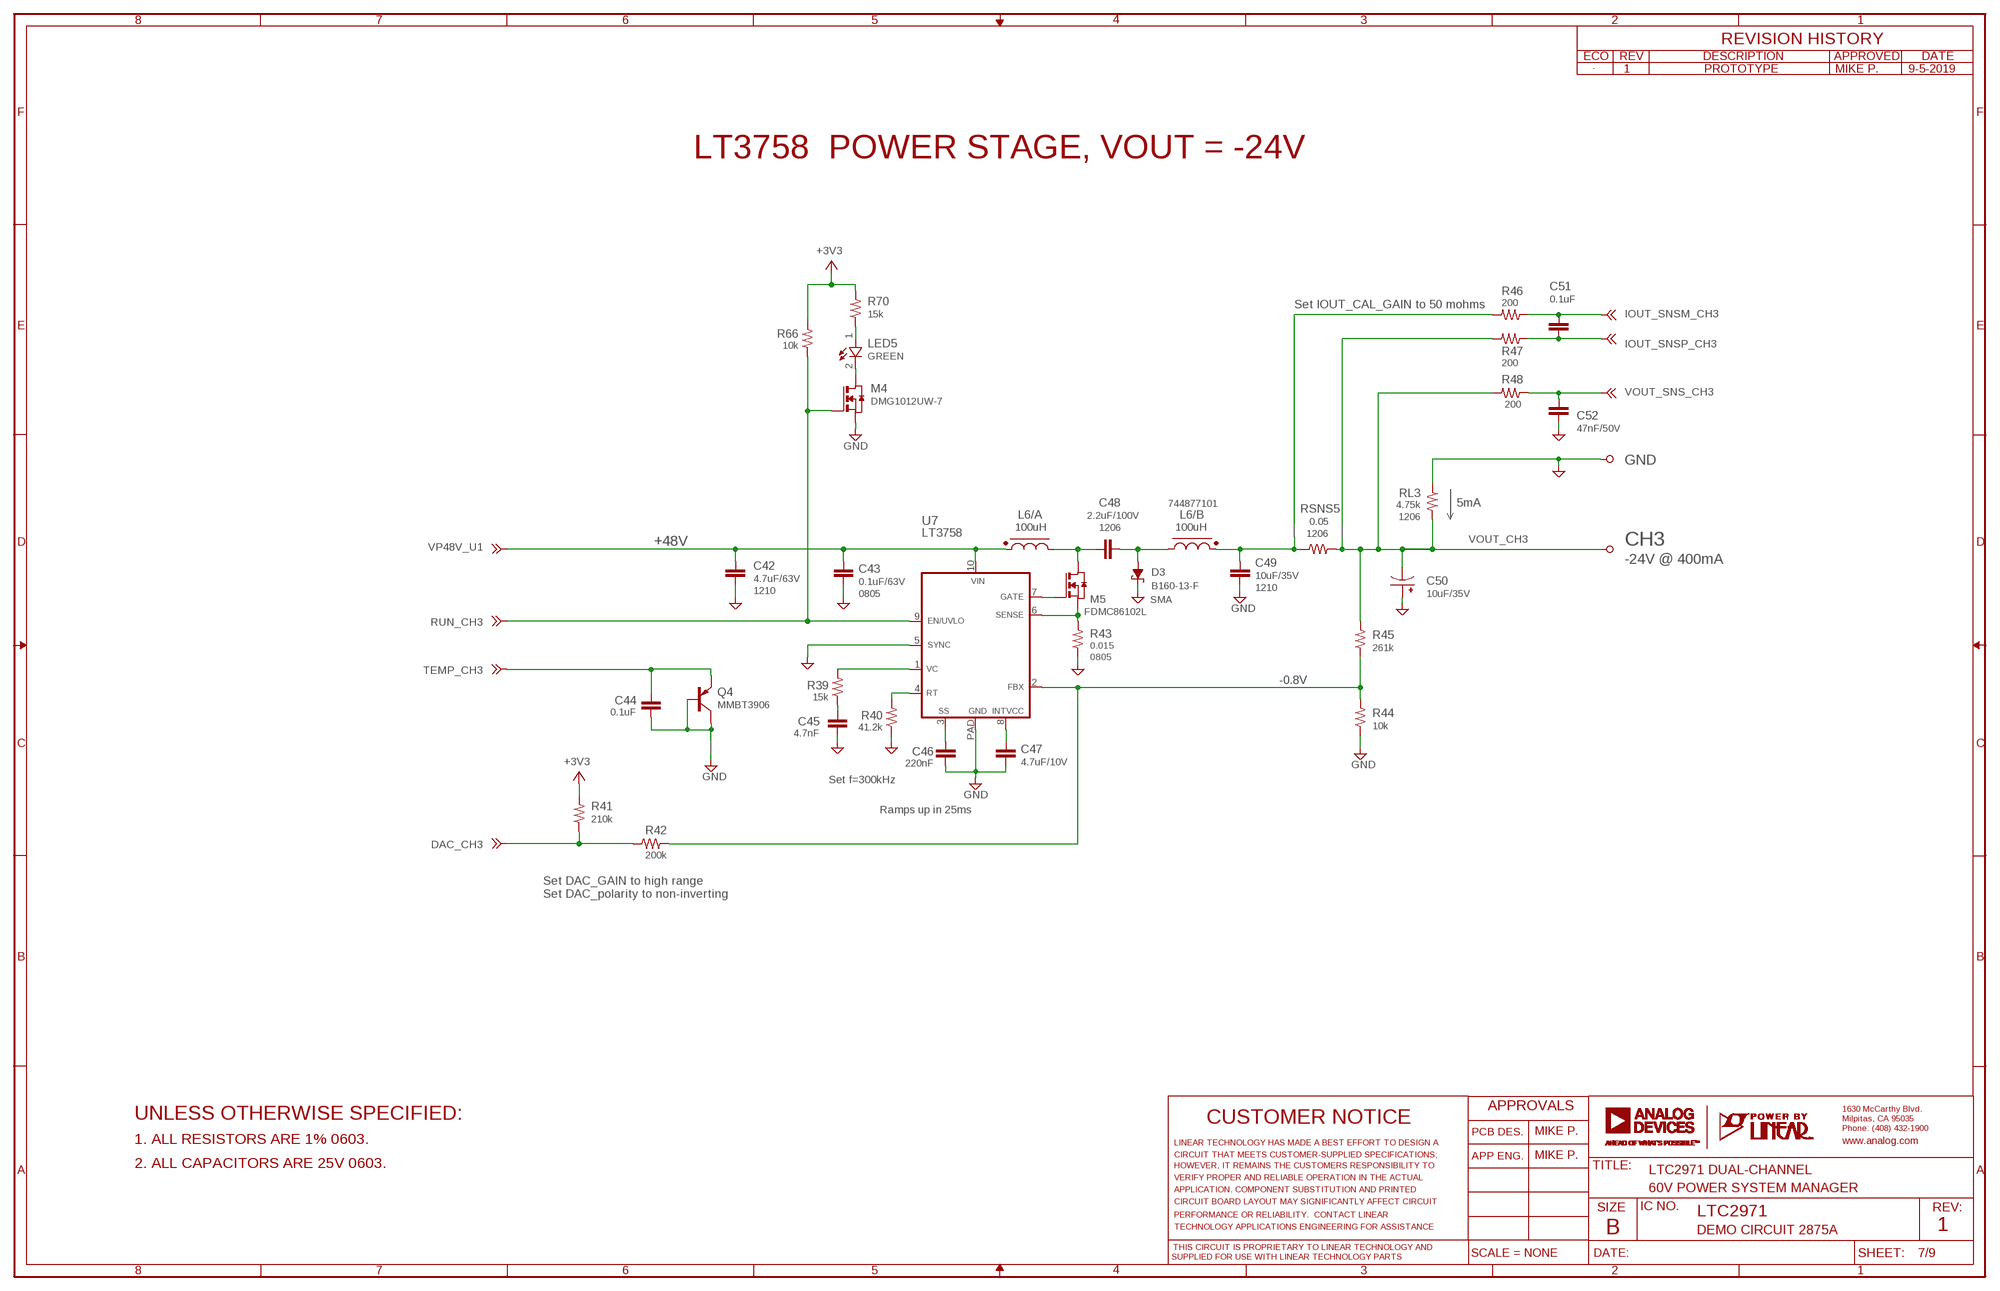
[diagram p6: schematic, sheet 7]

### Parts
C42  4.7uF/63V  CC1210_BOX  [C1210_BOX]
C43  0.1uF/63V  CC0805_BOX  [C0805_BOX]
C44  0.1uF  CC0603_BOX  [C0603_BOX]
C45  4.7nF  CC0603_BOX  [C0603_BOX]
C46  220nF  CC0603_BOX  [C0603_BOX]
C47  4.7uF/10V  CC0603_BOX  [C0603_BOX]
C48  2.2uF/100V  CC1206_BOX  [C1206_BOX]
C49  10uF/35V  CC1210_BOX  [C1210_BOX]
C50  10uF/35V  CPOL-USUD-6,3X5,8  [UD-6,3X5,8_NICHICON]
C51  0.1uF  CC0603_BOX  [C0603_BOX]
C52  47nF/50V  CC0603_BOX  [C0603_BOX]
D3  B160-13-F  SCHOTTKY-DIODESMA  [SMA]
L6  100uH  L_COUPLED_WURTH7.3  [WE-DD-7.3]
LED5  GREEN  LED-0603  [CHIPLED_0603]
M4  DMG1012UW-7  NCH(SOT323)  [SOT323]
M5  FDMC86102L  NCHMLP8  [MLP-8]
NB6  NODE_BREAKER  [NODE_BREAKER]
NB7  NODE_BREAKER  [NODE_BREAKER]
NB16  NODE_BREAKER  [NODE_BREAKER]
Q4  MMBT3906  PNP  [SC70]
R39  15k  RR0603_BOX  [R0603_BOX]
R40  41.2k  RR0603_BOX  [R0603_BOX]
R41  210k  RR0603_BOX  [R0603_BOX]
R42  200k  RR0603_BOX  [R0603_BOX]
R43  0.015  RR0805_BOX  [R0805_BOX]
R44  10k  RR0603_BOX  [R0603_BOX]
R45  261k  RR0603_BOX  [R0603_BOX]
R46  200  RR0603_BOX  [R0603_BOX]
R47  200  RR0603_BOX  [R0603_BOX]
R48  200  RR0603_BOX  [R0603_BOX]
R66  10k  RR0603_BOX  [R0603_BOX]
R70  15k  RR0603_BOX  [R0603_BOX]
RL3  4.75k  RR1206_BOX  [R1206_BOX]
RSNS5  0.05  RR1206_BOX  [R1206_BOX]
TP3  CH3  TURRET_LARGE_2501  [TURRET_LARGE_2501]
TP23  TURRET_SMALL_2308  [TURRET_SMALL_2308]
TP33  TESPOINT_SMD  TESTPOINT_SMDVIA  [VIA]
TP34  TESPOINT_SMD  TESTPOINT_SMDVIA  [VIA]
TP35  TESPOINT_SMD  TESTPOINT_SMDVIA  [VIA]
U7  LT3758  [MSOP10_EXP]

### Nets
DAC_CH3: R41.1 R42.1 TP35.1 ; also sheet 8
GND: C42.2 C43.2 C45.2 C46.2 C47.2 C49.2 C50.+ C52.2 D3.C M4.2(S) NB16.1 R40.1 R43.1 R44.1 RL3.1 TP23.TP1 U7.5(SYNC) U7.PAD(GND) ; also sheet 2,3,4,5,6,8,9
IOUT_SNSM_CH3: C51.1 R46.1 ; also sheet 8
IOUT_SNSP_CH3: C51.2 R47.1 ; also sheet 8
N$16: LED5.A R70.1
N$17: LED5.C M4.3(D)
N$22: M5.1(S) M5.2(S) M5.3(S) R43.2 U7.6(SENSE)
N$34: M5.4(G) U7.7(GATE)
N$42: C46.1 U7.3(SS)
N$43 [HV]: C48.1 L6.4 M5.5(D) M5.6(D) M5.7(D) M5.8(D) M5.PAD(D)
N$44 [HV]: C48.2 D3.A L6.3
N$45: R40.2 U7.4(RT)
N$47: R39.2 U7.1(VC)
N$50: C45.1 R39.1
N$62: C49.1 L6.2 NB6.1 RSNS5.1
N$69: C44.2 NB16.2 Q4.1(B) Q4.3(C)
N$77: C47.1 U7.8(INTVCC)
N$304: NB7.2 R47.2
N$305: NB6.2 R46.2
RUN_CH3: M4.1(G) R66.1 TP33.1 U7.9(EN/UVLO) ; also sheet 8
TEMP_CH3: C44.1 Q4.2(E) TP34.1 ; also sheet 8
VDD33_B: R41.2 R66.2 R70.2 ; supply symbol labelled +3V3 ; also sheet 6,8
VFB3: R42.2 R44.2 R45.1 U7.2(FBX)
VOUT_CH3: C50.- NB7.1 R45.2 R48.2 RL3.2 RSNS5.2 TP3.TP
VOUT_SNS_CH3: C52.1 R48.1 ; also sheet 8
VP48V_U1 [HV]: C42.1 C43.1 L6.1 U7.10(VIN) ; also sheet 2,6,8

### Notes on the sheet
- 1 | PROTOTYPE | MIKE P. | 9-5-2019
- LT3758  POWER STAGE, VOUT = -24V
- Set IOUT_CAL_GAIN to 50 mohms
- 744877101 | 5mA
- 1206
- 1206
- 1206
- +48V | CH3
- -24V @ 400mA
- 1210
- 1210
- 0805
- SMA
- 0805
- -0.8V
- Set f=300kHz
- Ramps up in 25ms
- Set DAC_GAIN to high range
  Set DAC_polarity to non-inverting
- UNLESS OTHERWISE SPECIFIED:
- MIKE P.
- 1. ALL RESISTORS ARE 1% 0603.
- MIKE P.
- 2. ALL CAPACITORS ARE 25V 0603.
- LTC2971 DUAL-CHANNEL
- 60V POWER SYSTEM MANAGER
- LTC2971
- DEMO CIRCUIT 2875A | 1

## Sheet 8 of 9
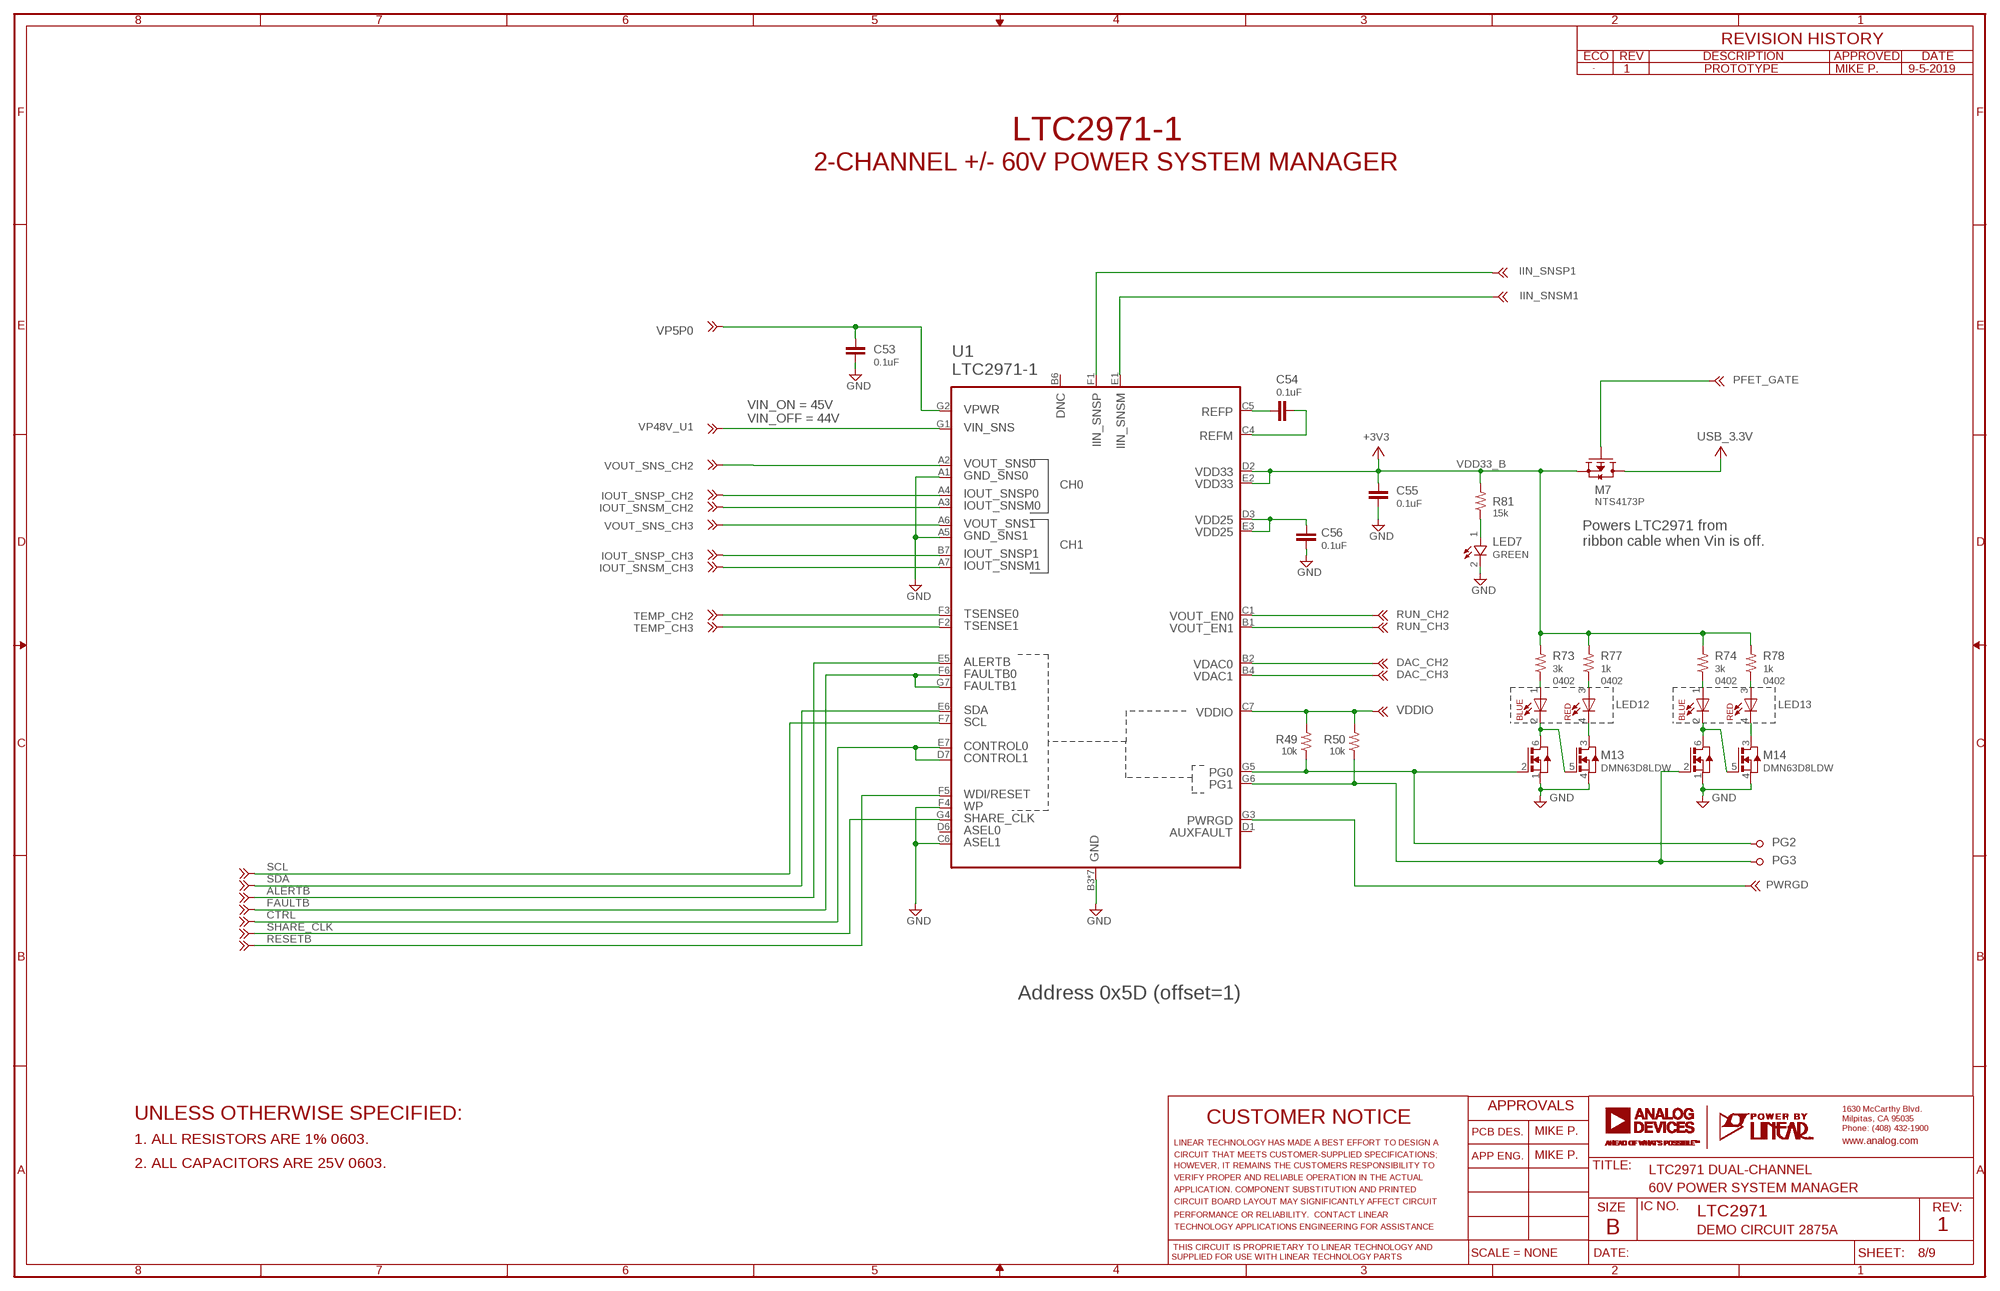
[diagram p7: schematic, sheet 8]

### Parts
C53  0.1uF  CC0603_BOX  [C0603_BOX]
C54  0.1uF  CC0603_BOX  [C0603_BOX]
C55  0.1uF  CC0603_BOX  [C0603_BOX]
C56  0.1uF  CC0603_BOX  [C0603_BOX]
LED7  GREEN  LED-0603  [CHIPLED_0603]
LED12  LED-DUAL-COLOR-BL-RD  [LED-DUAL_1.6X0.8MM]
LED13  LED-DUAL-COLOR-BL-RD  [LED-DUAL_1.6X0.8MM]
M7  NTS4173P  PCH(SOT323)  [SOT323]
M13  DMN63D8LDW  NCH_DUAL_REVERSIBLE  [SOT-363]
M14  DMN63D8LDW  NCH_DUAL_REVERSIBLE  [SOT-363]
R49  10k  RR0603_BOX  [R0603_BOX]
R50  10k  RR0603_BOX  [R0603_BOX]
R73  3k  RR0402_BOX  [R0402_BOX]
R74  3k  RR0402_BOX  [R0402_BOX]
R77  1k  RR0402_BOX  [R0402_BOX]
R78  1k  RR0402_BOX  [R0402_BOX]
R81  15k  RR0603_BOX  [R0603_BOX]
TP18  PG2  TURRET_SMALL_2308  [TURRET_SMALL_2308]
TP19  PG3  TURRET_SMALL_2308  [TURRET_SMALL_2308]
U1  LTC2971-1  LTC2971  [BGA49]

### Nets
ALERTB: U1.E5(ALERTB) ; also sheet 5,9
CTRL: U1.D7(CTRL1) U1.E7(CTRL0) ; also sheet 5,9
DAC_CH2: U1.B2(VDAC0) ; also sheet 6
DAC_CH3: U1.B4(VDAC1) ; also sheet 7
FAULTB: U1.F6(FAULTB0) U1.G7(FAULTB1) ; also sheet 5,9
GND: C53.2 C55.2 C56.2 LED7.C M13.1(S1) M13.4(S2) M14.1(S1) M14.4(S2) U1.A1(GND_SNS0) U1.A5(GND_SNS1) U1.B3(GND) U1.B5(GND) U1.C2(GND) U1.C3(GND) U1.C6(ASEL1) U1.D4(GND) U1.D5(GND) U1.E4(GND) U1.F4(WP) ; also sheet 2,3,4,5,6,7,9
IIN_SNSM1 [HV]: U1.E1(IIN_SNSM) ; also sheet 2
IIN_SNSP1 [HV]: U1.F1(IIN_SNSP) ; also sheet 2
IOUT_SNSM_CH2: U1.A3(IOUT_SNSM0) ; also sheet 6
IOUT_SNSM_CH3: U1.A7(IOUT_SNSM1) ; also sheet 7
IOUT_SNSP_CH2: U1.A4(IOUT_SNSP0) ; also sheet 6
IOUT_SNSP_CH3: U1.B7(IOUT_SNSP1) ; also sheet 7
N$14: C54.1 U1.C5(REFP)
N$15: C54.2 U1.C4(REFM)
N$19: C56.1 U1.D3(VDD25_IO) U1.E3(VDD25_IN)
N$65: LED7.A R81.1
N$84: LED12.2(C2) M13.5(G2) M13.6(D1)
N$85: LED12.4(C4) M13.3(D2)
N$86: LED13.2(C2) M14.5(G2) M14.6(D1)
N$87: LED13.4(C4) M14.3(D2)
N$88: LED13.1(A1) R74.1
N$89: LED13.3(A3) R78.1
N$91: LED12.1(A1) R73.1
N$92: LED12.3(A3) R77.1
PFET_GATE: M7.1(G) ; also sheet 5
PG2: M13.2(G1) R49.1 TP18.TP1 U1.G5(PG0)
PG3: M14.2(G1) R50.1 TP19.TP1 U1.G6(PG1)
PWRGD: U1.G3(PWRGD) ; also sheet 5,9
RESETB: U1.F5(WDI-RESET) ; also sheet 5,9
RUN_CH2: U1.C1(VOUT_EN0) ; also sheet 6
RUN_CH3: U1.B1(VOUT_EN1) ; also sheet 7
SCL: U1.F7(SCL) ; also sheet 5,9
SDA: U1.E6(SDA) ; also sheet 5,9
SHARE_CLK: U1.G4(SHARE_CLK) ; also sheet 5,9
TEMP_CH2: U1.F3(TSENSE0) ; also sheet 6
TEMP_CH3: U1.F2(TSENSE1) ; also sheet 7
USB_3.3V: M7.3(D) ; supply symbol labelled +3V3 ; also sheet 5,9
VDD33_B: C55.1 M7.2(S) R73.2 R74.2 R77.2 R78.2 R81.2 U1.D2(VDD33_IO) U1.E2(VDD33_IN) ; supply symbol labelled +3V3 ; also sheet 6,7
VDDIO: R49.2 R50.2 U1.C7(VDDIO) ; also sheet 5,9
VOUT_SNS_CH2: U1.A2(VOUT_SNS0) ; also sheet 6
VOUT_SNS_CH3: U1.A6(VOUT_SNS1) ; also sheet 7
VP5P0: C53.1 U1.G2(VPWR) ; also sheet 5
VP48V_U1 [HV]: U1.G1(VIN_SNS) ; also sheet 2,6,7
Unconnected: U1.B6(DNC) U1.D1(AUXFAULT) U1.D6(ASEL0)

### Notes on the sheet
- 1 | PROTOTYPE | MIKE P. | 9-5-2019
- LTC2971-1
- 2-CHANNEL +/- 60V POWER SYSTEM MANAGER
- VIN_ON = 45V
  VIN_OFF = 44V
- Powers LTC2971 from 
  ribbon cable when Vin is off.
- 0402 | 0402 | 0402 | 0402
- Address 0x5D (offset=1)
- UNLESS OTHERWISE SPECIFIED:
- MIKE P.
- 1. ALL RESISTORS ARE 1% 0603.
- MIKE P.
- 2. ALL CAPACITORS ARE 25V 0603.
- LTC2971 DUAL-CHANNEL
- 60V POWER SYSTEM MANAGER
- LTC2971
- DEMO CIRCUIT 2875A | 1

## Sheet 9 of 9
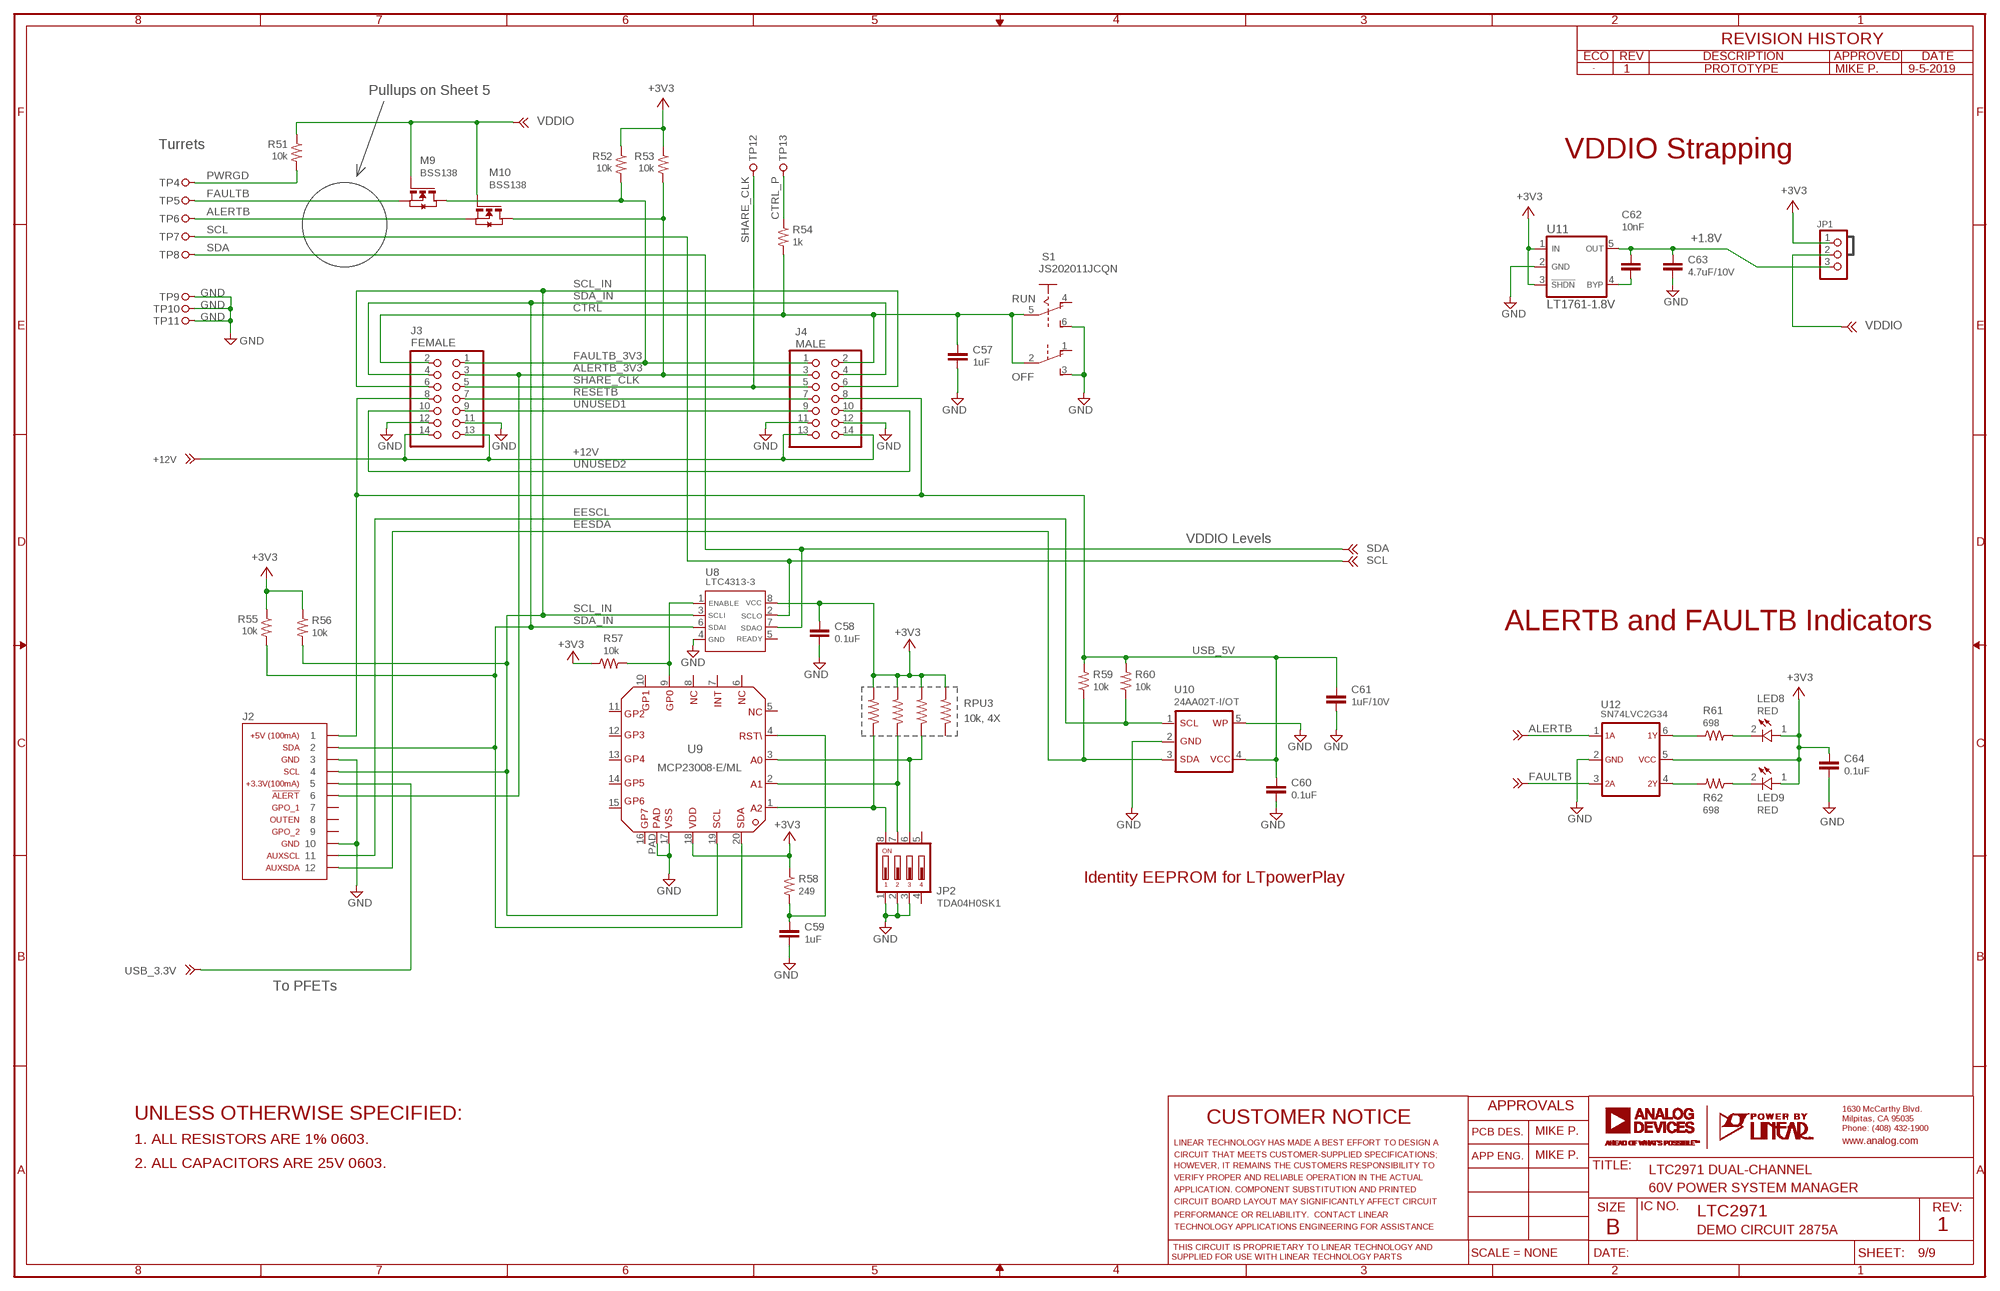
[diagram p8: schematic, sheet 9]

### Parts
C57  1uF  CC0603_BOX  [C0603_BOX]
C58  0.1uF  CC0603_BOX  [C0603_BOX]
C59  1uF  CC0603_BOX  [C0603_BOX]
C60  0.1uF  CC0603_BOX  [C0603_BOX]
C61  1uF/10V  CC0603_BOX  [C0603_BOX]
C62  10nF  CC0603_BOX  [C0603_BOX]
C63  4.7uF/10V  CC0603_BOX  [C0603_BOX]
C64  0.1uF  CC0603_BOX  [C0603_BOX]
J2  CONN_DC1613_STD  [CONN_DC1613]
J3  FEMALE  PINHD-2X07_2.00  [2X07M]
J4  MALE  PINHD-2X07_2.00  [2X07M]
JP1  PINHD-1X3-2MM  [1X03-2MM]
JP2  TDA04H0SK1  [SMT_DIP_4]
LED8  RED  LED-0603  [CHIPLED_0603]
LED9  RED  LED-0603  [CHIPLED_0603]
M9  BSS138  NCH(SOT323)  [SOT323]
M10  BSS138  NCH(SOT323)  [SOT323]
R51  10k  RR0603_BOX  [R0603_BOX]
R52  10k  RR0603_BOX  [R0603_BOX]
R53  10k  RR0603_BOX  [R0603_BOX]
R54  1k  RR0603_BOX  [R0603_BOX]
R55  10k  RR0603_BOX  [R0603_BOX]
R56  10k  RR0603_BOX  [R0603_BOX]
R57  10k  RR0603_BOX  [R0603_BOX]
R58  249  RR0603_BOX  [R0603_BOX]
R59  10k  RR0603_BOX  [R0603_BOX]
R60  10k  RR0603_BOX  [R0603_BOX]
R61  698  RR0603_BOX  [R0603_BOX]
R62  698  RR0603_BOX  [R0603_BOX]
RPU3  10k, 4X  R_ARRAY_4X_CRA06S  [R_VISHAY_CRA06S]
S1  JS202011JCQN  [JCQN]
TP4  PWRGD  TURRET_LARGE_2501  [TURRET_LARGE_2501]
TP5  FAULT  TURRET_LARGE_2501  [TURRET_LARGE_2501]
TP6  ALERT  TURRET_LARGE_2501  [TURRET_LARGE_2501]
TP7  SCL  TURRET_LARGE_2501  [TURRET_LARGE_2501]
TP8  SDA  TURRET_LARGE_2501  [TURRET_LARGE_2501]
TP9  GND  TURRET_LARGE_2501  [TURRET_LARGE_2501]
TP10  GND  TURRET_LARGE_2501  [TURRET_LARGE_2501]
TP11  GND  TURRET_LARGE_2501  [TURRET_LARGE_2501]
TP12  SHARE_CLK  TURRET_LARGE_2501  [TURRET_LARGE_2501]
TP13  CTRL  TURRET_LARGE_2501  [TURRET_LARGE_2501]
U8  LTC4313-3  LTC4313_MS8  [MSOP-8]
U9  MCP23008-E/ML  [QFN20]
U10  24AA02T-I/OT  24AA64  [SOT-23-5]
U11  LT1761-1.8V  LT1761-X  [SOT-23-5]
U12  SN74LVC2G34  [SC70-6]

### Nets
+12V: J3.13 J3.14 J4.13 J4.14 ; also sheet 2
A0_MUX: JP2.6 RPU3.R2_1 U9.3
A1_MUX: JP2.7 RPU3.R3_1 U9.2
A2_MUX: JP2.8 RPU3.R4_1 U9.1
ALERTB: M10.2(S) TP6.TP U12.1 ; also sheet 5,8
ALERTB_3V3: J2.6 J3.3 J4.3 M10.3(D) R53.2
CTRL: C57.1 J3.2 J4.2 R54.2 S1.2(B:P) S1.5(A:P) ; also sheet 5,8
CTRL_P: R54.1 TP13.TP
EESCL: J2.11 R60.1 U10.1
EESDA: J2.12 R59.1 U10.3
FAULTB: M9.2(S) TP5.TP U12.3 ; also sheet 5,8
FAULTB_3V3: J3.1 J4.1 M9.3(D) R52.2
GND: C57.2 C58.2 C59.2 C60.2 C61.2 C63.2 C64.2 J2.3 J2.10 J3.11 J3.12 J4.11 J4.12 JP2.1 JP2.2 JP2.3 S1.3(B:S) S1.6(A:S) TP9.TP TP10.TP TP11.TP U8.4(GND) U9.17 U9.PAD U10.2 U10.5 U11.2(GND) U12.2 ; also sheet 2,3,4,5,6,7,8
N$1: R61.1 U12.6
N$3: LED8.C R61.2
N$24: C62.2 U11.4(BYP)
N$25: R62.2 U12.4
N$26: LED9.C R62.1
N$54: C62.1 C63.1 JP1.3 U11.5(OUT)
N$66: C59.1 R58.2 U9.4
N$74: R57.2 U8.1(EN) U9.9
PWRGD: R51.2 TP4.TP ; also sheet 5,8
RESETB: J3.7 J4.7 ; also sheet 5,8
SCL: TP7.TP U8.2(SCLO) ; also sheet 5,8
SCL_IN: J2.4 J3.6 J4.6 R56.2 U8.3(SCLI) U9.19
SDA: TP8.TP U8.7(SDAO) ; also sheet 5,8
SDA_IN: J2.2 J3.4 J4.4 R55.2 U8.6(SDAI) U9.20
SHARE_CLK: J3.5 J4.5 TP12.TP ; also sheet 5,8
UNUSED1: J3.9 J4.9
UNUSED2: J3.10 J4.10
USB_3.3V: J2.5 ; also sheet 5,8
USB_5V: C60.1 C61.1 J2.1 J3.8 J4.8 R59.2 R60.2 U10.4
VDD33_A: C58.1 C64.1 JP1.1 LED8.A LED9.A R52.1 R53.1 R55.1 R56.1 R57.1 R58.1 RPU3.R1_2 RPU3.R2_2 RPU3.R3_2 RPU3.R4_2 U8.8(VCC) U9.18 U11.1(IN) U11.3(SHDN) U12.5 ; supply symbol labelled +3V3 ; also sheet 3,4,5,6
VDDIO: JP1.2 M9.1(G) M10.1(G) R51.1 ; also sheet 5,8
Unconnected: J2.7 J2.8 J2.9 JP2.4 JP2.5 RPU3.R1_1 S1.1(B:O) S1.4(A:O) U8.5(RDY) U9.5 U9.6 U9.7 U9.8 U9.10 U9.11 U9.12 U9.13 U9.14 U9.15 U9.16

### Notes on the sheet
- 1 | PROTOTYPE | MIKE P. | 9-5-2019
- Pullups on Sheet 5
- Turrets
- VDDIO Strapping
- +1.8V
- RUN
- OFF
- VDDIO Levels
- ALERTB and FAULTB Indicators
- Identity EEPROM for LTpowerPlay
- To PFETs
- UNLESS OTHERWISE SPECIFIED:
- MIKE P.
- 1. ALL RESISTORS ARE 1% 0603.
- MIKE P.
- 2. ALL CAPACITORS ARE 25V 0603.
- LTC2971 DUAL-CHANNEL
- 60V POWER SYSTEM MANAGER
- LTC2971
- DEMO CIRCUIT 2875A | 1

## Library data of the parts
C1 C13 C21 C39 C50 = rcl:CPOL-US: POLARIZED CAPACITOR, American symbol
C2-C12 C14-C20 C22-C38 C40-C49 C51-C64 = rcl:C: CAPACITOR, European symbol
D1-D3 = diode:SCHOTTKY-DIODE: Schottky Diode
J1 = power-jack:PJ-002A: DC Power Jack, 2.5A, 2.0mm ID, 5.5mm OD
J2 = con-fci:CONN_DC1613: Connector for LT DC1613 USB Dongle
J3 = pinhead_2mm:PINHD-2X07: PIN HEADER
J4 = pinhead-2mm:PINHD-2X07: PIN HEADER
JP1 = pinhead:PINHD-1X3-2MM: PIN HEADER
JP2 = kalin:TDA04H0SK1: Ultra-miniature Surface Mount Half-pitch DIP Switch
L1-L5 = inductors:L: Inductor
L6 = inductors:L_COUPLED_WURTH
LED1-LED9 = led:LED-0603: SMD LED in R0603
LED10-LED13 = led:LED-DUAL-COLOR-BL-RD
M1-M5 M8-M10 = transistor-fet:NCH
M6 M7 = transistor-fet:PCH
M11-M14 = transistor-fet:NCH_DUAL_REVERSIBLE
NB1-NB7 NB14-NB16 NB19-NB21 = solderpad:NODE_BREAKER: NODE BREAKER (top layer)
NB12 NB13 NB17 NB18 = solderpad:NODE_BREAKER_BOT: NODE BREAKER (bottom layer)
Q1-Q4 = transistor-small-signal:PNP
R1-R82 RL0 RL1-RL3 RSNS0 RSNS1-RSNS5 = resistor:R: RESISTOR, American symbol
RPU1-RPU3 = resistor:R_ARRAY_4X_CRA06S: Thick Film Resistor Array
S1 = switch:JS202011: SLIDING SWITCH Siemens, distributor Buerklin, 11G766
SW1 SW2 = kalin:SWITCH_PTS635: PTS635SL25 Surface Mount Tactile Switch
TP0 TP1-TP15 = testpad:TURRET_LARGE_2501: Large Test Turret Mill Max 2501
TP16-TP23 = testpad:TURRET_SMALL_2308: Small Test Turret Mill-Max 2308
TP24-TP36 = testpad:TESTPOINT_SMD: Small SMD Test Point
U0 U1 = linear-technology:LTC2971: 2-Ch +/- 60V Power System Manager with EEPROM (BGA49)
U2 = linear-technology:LT3958: 80V, 3.3A, Boost, Flyback, SEPIC, Inverting Converter
U3 = linear-technology:LT7101: 105V 1A Sync Step-Down Regulator with Fast Current Programming
U4 = linear-technology:LT3991
U5 = analog-devices:ADP2360
U6 = linear-technology:LT8630: 100V, 0.6A Synchronous Micropower Step-Down High Efficiency Switching Regulator
U7 = linear-technology:LT3758: 100V Input Boost, SEPIC, Inverting Controller
U8 = linear-technology:LTC4313: 2-Wire Bus Buffers with High Noise Margin
U9 = kalin:MCP23008: I2C 8-pin IO Expander
U10 = kalin:24AA64: 64Kbit I2C Serial EEPROM in SOT-23-5
U11 = linear-technology:LT1761-X: 100mA, Low Noise, Fixed LDO Micropower Regulators w/ SHDN in TSOT-23
U12 = kalin:SN74LVC2G34: Dual Buffer Gate

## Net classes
1 HV: clearance 0.178 mm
